//FC651	Send/Receive Schnittstelle
// ***************************************************************************
FUNCTION "FC_SR_QK" : VOID

TITLE =Send/Receive Empfang

AUTHOR: 	SIEMENS
FAMILY: 	SISTARS7
VERSION: 	4.02

//KNOW_HOW_PROTECT

// Datum	 Name			Aktion
// ---------------------------------------------------------------------------
// 19.05.99  Mahler		Neu



//Eingabeparameter
VAR_INPUT
	iFKT			: INT;		//Aufrufmodus
END_VAR

//Ausgabeparameter
//VAR_OUTPUT
//END_VAR


//Temporäre/Lokale Variable
VAR_TEMP

	anyQUEL	: ANY; 	         //Offset=0, Zeiger muss an erster Stelle stehen
	anyZIEL	: ANY;		   //Offset=10,
	uVerb		:"XC_INIT_SR_UDT";   //Offset=20


	iID		: INT;
	wLADDR	: WORD;

	boNDR		: BOOL;
	boDONE	: BOOL;
	boERROR	: BOOL;
	wSTATUS	: WORD;
	iLEN		: INT;

	iret		: INT;

 	iLoop	      : INT;
      iAct		: INT;

	dwPTR1      : DWORD;
	dwPTR2	: DWORD;
      dwOff		: DWORD;

	boSend	: BOOL;

	byPCU		: BYTE;
	bySavVB	: BYTE;

	bosec		: BOOL;
	bomin		: BOOL;
	iTSoll	: INT;
	iTIst		: INT;

END_VAR

BEGIN

NETWORK
TITLE = Vorbesetzen der Zeiger
// ===========================================================================
//Pionter fuer den Empfangspuffer zusammenstellen
//Any-Pointer:
//Byte 0	: S7-Typ 		= 16=10H                 LB0,LB10
//Byte 1	: Datentyp		= 02=Byte			 LB1,LB11
//Byte 2/3	: Wiederholungsfaktor				 LW2,LW12
//Byte 4/5	: DB-Nummer						 LW4,LW14
//Byte 6-9	: Bereichszeiger					 LD6,LD16

	L 16;		//S7-Typ
	T LB 0;
	T LB 10;
	L 2;		//Datentyp=Byte
	T LB1;
	T LB11;

	L "SYS".u.byAS;
      T  #byPCU;
	L "XC_VERB_SR".bPCU;		//Pruefen ob PCU-NR im Bereich 1 .. 16 veraendert
	==I;
      spb end1;
	l #byPCU;
	l 16;
	>I;
	spb end1;
	l #byPCU;
	T "XC_VERB_SR".bPCU;
      S "XC_VERB_SR".boINIT;
end1: nop 0;
NETWORK
TITLE =INIT	- Verbindungsblock vorbesetzen
// ===========================================================================
      l iFKT;
      l 1;
      <>I;
	spb end2;
	un "XC_VERB_SR".boINIT;
      SPB end2;
      R "XC_VERB_SR".boINIT;

//PCU-Nummer je nach eigener Nummer eintragen
      L  "XC_VERB_SR".iOffset;
      L 1;
      +I;
      sld 3;
      t #dwPtr1;						//Zeiger auf DBB fuer PCU z.B. 201 Aktiv
      L  "XC_VERB_SR".iOffset;
      L 7;
      +I;
      sld 3;
      t #dwPtr2;						//Zeiger auf DBB fuer PCU z.B. 207 Normal
      L  "XC_VERB_SR".iLen;
      sld 3;
	t #dwOff;

	AUF "XC_VERB_SR";

      L  #byPCU;			//Sprungleiste
      spl ende;
      spa Lo20;
      spa AS01;
      spa AS02;
      spa AS03;
      spa AS04;
      spa AS05;
      spa AS06;
      spa AS07;
      spa AS08;
      spa AS09;
      spa AS10;
      spa AS11;
      spa AS12;
      spa AS13;
      spa AS14;
      spa AS15;
      spa AS16;
ende:	spa Lo20;

AS01:	L 2; 							//Verbindung 1 PCU-NR eintragen
    	T  DBB[#dwPTR1];
	T  DBB[#dwPTR2];
      L  #dwOff;
      L  #dwPTR1;
      +D;
      T  #dwPTR1;
      L  #dwOff;
      L  #dwPTR2;
      +D;
      T  #dwPTR2;

	L 3; 							//Verbindung 2 PCU-NR eintragen
    	T  DBB[#dwPTR1];
	T  DBB[#dwPTR2];
      L  #dwOff;
      L  #dwPTR1;
      +D;
      T  #dwPTR1;
      L  #dwOff;
      L  #dwPTR2;
      +D;
      T  #dwPTR2;

	L 4; 							//Verbindung 3 PCU-NR eintragen
    	T  DBB[#dwPTR1];
	T  DBB[#dwPTR2];
      L  #dwOff;
      L  #dwPTR1;
      +D;
      T  #dwPTR1;
      L  #dwOff;
      L  #dwPTR2;
      +D;
      T  #dwPTR2;

	L 5; 							//Verbindung 4 PCU-NR eintragen
    	T  DBB[#dwPTR1];
	T  DBB[#dwPTR2];
      L  #dwOff;
      L  #dwPTR1;
      +D;
      T  #dwPTR1;
      L  #dwOff;
      L  #dwPTR2;
      +D;
      T  #dwPTR2;

	L 6; 							//Verbindung 5 PCU-NR eintragen
    	T  DBB[#dwPTR1];
	T  DBB[#dwPTR2];
      L  #dwOff;
      L  #dwPTR1;
      +D;
      T  #dwPTR1;
      L  #dwOff;
      L  #dwPTR2;
      +D;
      T  #dwPTR2;


	L 7; 							//Verbindung 6 PCU-NR eintragen
    	T  DBB[#dwPTR1];
	T  DBB[#dwPTR2];
      L  #dwOff;
      L  #dwPTR1;
      +D;
      T  #dwPTR1;
      L  #dwOff;
      L  #dwPTR2;
      +D;
      T  #dwPTR2;

	L 8; 							//Verbindung 7 PCU-NR eintragen
    	T  DBB[#dwPTR1];
	T  DBB[#dwPTR2];
      L  #dwOff;
      L  #dwPTR1;
      +D;
      T  #dwPTR1;
      L  #dwOff;
      L  #dwPTR2;
      +D;
      T  #dwPTR2;

	L 9; 							//Verbindung 8  PCU-NR eintragen
    	T  DBB[#dwPTR1];
	T  DBB[#dwPTR2];
      L  #dwOff;
      L  #dwPTR1;
      +D;
      T  #dwPTR1;
      L  #dwOff;
      L  #dwPTR2;
      +D;
      T  #dwPTR2;

	L 10; 						//Verbindung 9 PCU-NR eintragen
    	T  DBB[#dwPTR1];
	T  DBB[#dwPTR2];
      L  #dwOff;
      L  #dwPTR1;
      +D;
      T  #dwPTR1;
      L  #dwOff;
      L  #dwPTR2;
      +D;
      T  #dwPTR2;

	L 11; 						//Verbindung 10 PCU-NR eintragen
    	T  DBB[#dwPTR1];
	T  DBB[#dwPTR2];
      L  #dwOff;
      L  #dwPTR1;
      +D;
      T  #dwPTR1;
      L  #dwOff;
      L  #dwPTR2;
      +D;
      T  #dwPTR2;

	L 12; 						//Verbindung 11 PCU-NR eintragen
    	T  DBB[#dwPTR1];
	T  DBB[#dwPTR2];
      L  #dwOff;
      L  #dwPTR1;
      +D;
      T  #dwPTR1;
      L  #dwOff;
      L  #dwPTR2;
      +D;
      T  #dwPTR2;

	L 13; 						//Verbindung 12 PCU-NR eintragen
    	T  DBB[#dwPTR1];
	T  DBB[#dwPTR2];
      L  #dwOff;
      L  #dwPTR1;
      +D;
      T  #dwPTR1;
      L  #dwOff;
      L  #dwPTR2;
      +D;
      T  #dwPTR2;

	L 14; 						//Verbindung 13 PCU-NR eintragen
    	T  DBB[#dwPTR1];
	T  DBB[#dwPTR2];
      L  #dwOff;
      L  #dwPTR1;
      +D;
      T  #dwPTR1;
      L  #dwOff;
      L  #dwPTR2;
      +D;
      T  #dwPTR2;

	L 15; 						//Verbindung 14 PCU-NR eintragen
    	T  DBB[#dwPTR1];
	T  DBB[#dwPTR2];
      L  #dwOff;
      L  #dwPTR1;
      +D;
      T  #dwPTR1;
      L  #dwOff;
      L  #dwPTR2;
      +D;
      T  #dwPTR2;

	L 16; 						//Verbindung 15 PCU-NR eintragen
    	T  DBB[#dwPTR1];
	T  DBB[#dwPTR2];
      L  #dwOff;
      L  #dwPTR1;
      +D;
      T  #dwPTR1;
      L  #dwOff;
      L  #dwPTR2;
      +D;
      T  #dwPTR2;
	spa Lo20;

AS02:	L 1; 							//Verbindung 1 PCU-NR eintragen
    	T  DBB[#dwPTR1];
	T  DBB[#dwPTR2];
      L  #dwOff;
      L  #dwPTR1;
      +D;
      T  #dwPTR1;
      L  #dwOff;
      L  #dwPTR2;
      +D;
      T  #dwPTR2;

	L 16; 							//Verbindung 2 PCU-NR eintragen
    	T  DBB[#dwPTR1];
	T  DBB[#dwPTR2];
      L  #dwOff;
      L  #dwPTR1;
      +D;
      T  #dwPTR1;
      L  #dwOff;
      L  #dwPTR2;
      +D;
      T  #dwPTR2;

	L 3; 							//Verbindung 3 PCU-NR eintragen
    	T  DBB[#dwPTR1];
	T  DBB[#dwPTR2];
      L  #dwOff;
      L  #dwPTR1;
      +D;
      T  #dwPTR1;
      L  #dwOff;
      L  #dwPTR2;
      +D;
      T  #dwPTR2;

	L 4; 							//Verbindung 4 PCU-NR eintragen
    	T  DBB[#dwPTR1];
	T  DBB[#dwPTR2];
      L  #dwOff;
      L  #dwPTR1;
      +D;
      T  #dwPTR1;
      L  #dwOff;
      L  #dwPTR2;
      +D;
      T  #dwPTR2;

	L 5; 							//Verbindung 5 PCU-NR eintragen
    	T  DBB[#dwPTR1];
	T  DBB[#dwPTR2];
      L  #dwOff;
      L  #dwPTR1;
      +D;
      T  #dwPTR1;
      L  #dwOff;
      L  #dwPTR2;
      +D;
      T  #dwPTR2;


	L 6; 							//Verbindung 6 PCU-NR eintragen
    	T  DBB[#dwPTR1];
	T  DBB[#dwPTR2];
      L  #dwOff;
      L  #dwPTR1;
      +D;
      T  #dwPTR1;
      L  #dwOff;
      L  #dwPTR2;
      +D;
      T  #dwPTR2;

	L 7; 							//Verbindung 7 PCU-NR eintragen
    	T  DBB[#dwPTR1];
	T  DBB[#dwPTR2];
      L  #dwOff;
      L  #dwPTR1;
      +D;
      T  #dwPTR1;
      L  #dwOff;
      L  #dwPTR2;
      +D;
      T  #dwPTR2;

	L 8; 							//Verbindung 8  PCU-NR eintragen
    	T  DBB[#dwPTR1];
	T  DBB[#dwPTR2];
      L  #dwOff;
      L  #dwPTR1;
      +D;
      T  #dwPTR1;
      L  #dwOff;
      L  #dwPTR2;
      +D;
      T  #dwPTR2;

	L 9; 						//Verbindung 9 PCU-NR eintragen
    	T  DBB[#dwPTR1];
	T  DBB[#dwPTR2];
      L  #dwOff;
      L  #dwPTR1;
      +D;
      T  #dwPTR1;
      L  #dwOff;
      L  #dwPTR2;
      +D;
      T  #dwPTR2;

	L 10; 						//Verbindung 10 PCU-NR eintragen
    	T  DBB[#dwPTR1];
	T  DBB[#dwPTR2];
      L  #dwOff;
      L  #dwPTR1;
      +D;
      T  #dwPTR1;
      L  #dwOff;
      L  #dwPTR2;
      +D;
      T  #dwPTR2;

	L 11; 						//Verbindung 11 PCU-NR eintragen
    	T  DBB[#dwPTR1];
	T  DBB[#dwPTR2];
      L  #dwOff;
      L  #dwPTR1;
      +D;
      T  #dwPTR1;
      L  #dwOff;
      L  #dwPTR2;
      +D;
      T  #dwPTR2;

	L 12; 						//Verbindung 12 PCU-NR eintragen
    	T  DBB[#dwPTR1];
	T  DBB[#dwPTR2];
      L  #dwOff;
      L  #dwPTR1;
      +D;
      T  #dwPTR1;
      L  #dwOff;
      L  #dwPTR2;
      +D;
      T  #dwPTR2;

	L 13; 						//Verbindung 13 PCU-NR eintragen
    	T  DBB[#dwPTR1];
	T  DBB[#dwPTR2];
      L  #dwOff;
      L  #dwPTR1;
      +D;
      T  #dwPTR1;
      L  #dwOff;
      L  #dwPTR2;
      +D;
      T  #dwPTR2;

	L 14; 						//Verbindung 14 PCU-NR eintragen
    	T  DBB[#dwPTR1];
	T  DBB[#dwPTR2];
      L  #dwOff;
      L  #dwPTR1;
      +D;
      T  #dwPTR1;
      L  #dwOff;
      L  #dwPTR2;
      +D;
      T  #dwPTR2;

	L 15; 						//Verbindung 15 PCU-NR eintragen
    	T  DBB[#dwPTR1];
	T  DBB[#dwPTR2];
      L  #dwOff;
      L  #dwPTR1;
      +D;
      T  #dwPTR1;
      L  #dwOff;
      L  #dwPTR2;
      +D;
      T  #dwPTR2;
	spa Lo20;

AS03:	L 15; 							//Verbindung 1 PCU-NR eintragen
    	T  DBB[#dwPTR1];
	T  DBB[#dwPTR2];
      L  #dwOff;
      L  #dwPTR1;
      +D;
      T  #dwPTR1;
      L  #dwOff;
      L  #dwPTR2;
      +D;
      T  #dwPTR2;

	L 1; 							//Verbindung 2 PCU-NR eintragen
    	T  DBB[#dwPTR1];
	T  DBB[#dwPTR2];
      L  #dwOff;
      L  #dwPTR1;
      +D;
      T  #dwPTR1;
      L  #dwOff;
      L  #dwPTR2;
      +D;
      T  #dwPTR2;

	L 2; 							//Verbindung 3 PCU-NR eintragen
    	T  DBB[#dwPTR1];
	T  DBB[#dwPTR2];
      L  #dwOff;
      L  #dwPTR1;
      +D;
      T  #dwPTR1;
      L  #dwOff;
      L  #dwPTR2;
      +D;
      T  #dwPTR2;

	L 16; 							//Verbindung 4 PCU-NR eintragen
    	T  DBB[#dwPTR1];
	T  DBB[#dwPTR2];
      L  #dwOff;
      L  #dwPTR1;
      +D;
      T  #dwPTR1;
      L  #dwOff;
      L  #dwPTR2;
      +D;
      T  #dwPTR2;

	L 4; 							//Verbindung 5 PCU-NR eintragen
    	T  DBB[#dwPTR1];
	T  DBB[#dwPTR2];
      L  #dwOff;
      L  #dwPTR1;
      +D;
      T  #dwPTR1;
      L  #dwOff;
      L  #dwPTR2;
      +D;
      T  #dwPTR2;


	L 5; 							//Verbindung 6 PCU-NR eintragen
    	T  DBB[#dwPTR1];
	T  DBB[#dwPTR2];
      L  #dwOff;
      L  #dwPTR1;
      +D;
      T  #dwPTR1;
      L  #dwOff;
      L  #dwPTR2;
      +D;
      T  #dwPTR2;

	L 6; 							//Verbindung 7 PCU-NR eintragen
    	T  DBB[#dwPTR1];
	T  DBB[#dwPTR2];
      L  #dwOff;
      L  #dwPTR1;
      +D;
      T  #dwPTR1;
      L  #dwOff;
      L  #dwPTR2;
      +D;
      T  #dwPTR2;

	L 7; 							//Verbindung 8  PCU-NR eintragen
    	T  DBB[#dwPTR1];
	T  DBB[#dwPTR2];
      L  #dwOff;
      L  #dwPTR1;
      +D;
      T  #dwPTR1;
      L  #dwOff;
      L  #dwPTR2;
      +D;
      T  #dwPTR2;

	L 8; 						//Verbindung 9 PCU-NR eintragen
    	T  DBB[#dwPTR1];
	T  DBB[#dwPTR2];
      L  #dwOff;
      L  #dwPTR1;
      +D;
      T  #dwPTR1;
      L  #dwOff;
      L  #dwPTR2;
      +D;
      T  #dwPTR2;

	L 9; 						//Verbindung 10 PCU-NR eintragen
    	T  DBB[#dwPTR1];
	T  DBB[#dwPTR2];
      L  #dwOff;
      L  #dwPTR1;
      +D;
      T  #dwPTR1;
      L  #dwOff;
      L  #dwPTR2;
      +D;
      T  #dwPTR2;

	L 10; 						//Verbindung 11 PCU-NR eintragen
    	T  DBB[#dwPTR1];
	T  DBB[#dwPTR2];
      L  #dwOff;
      L  #dwPTR1;
      +D;
      T  #dwPTR1;
      L  #dwOff;
      L  #dwPTR2;
      +D;
      T  #dwPTR2;

	L 11; 						//Verbindung 12 PCU-NR eintragen
    	T  DBB[#dwPTR1];
	T  DBB[#dwPTR2];
      L  #dwOff;
      L  #dwPTR1;
      +D;
      T  #dwPTR1;
      L  #dwOff;
      L  #dwPTR2;
      +D;
      T  #dwPTR2;

	L 12; 						//Verbindung 13 PCU-NR eintragen
    	T  DBB[#dwPTR1];
	T  DBB[#dwPTR2];
      L  #dwOff;
      L  #dwPTR1;
      +D;
      T  #dwPTR1;
      L  #dwOff;
      L  #dwPTR2;
      +D;
      T  #dwPTR2;

	L 13; 						//Verbindung 14 PCU-NR eintragen
    	T  DBB[#dwPTR1];
	T  DBB[#dwPTR2];
      L  #dwOff;
      L  #dwPTR1;
      +D;
      T  #dwPTR1;
      L  #dwOff;
      L  #dwPTR2;
      +D;
      T  #dwPTR2;

	L 14; 						//Verbindung 15 PCU-NR eintragen
    	T  DBB[#dwPTR1];
	T  DBB[#dwPTR2];
      L  #dwOff;
      L  #dwPTR1;
      +D;
      T  #dwPTR1;
      L  #dwOff;
      L  #dwPTR2;
      +D;
      T  #dwPTR2;
	spa Lo20;

AS04:	L 14; 							//Verbindung 1 PCU-NR eintragen
    	T  DBB[#dwPTR1];
	T  DBB[#dwPTR2];
      L  #dwOff;
      L  #dwPTR1;
      +D;
      T  #dwPTR1;
      L  #dwOff;
      L  #dwPTR2;
      +D;
      T  #dwPTR2;

	L 15; 							//Verbindung 2 PCU-NR eintragen
    	T  DBB[#dwPTR1];
	T  DBB[#dwPTR2];
      L  #dwOff;
      L  #dwPTR1;
      +D;
      T  #dwPTR1;
      L  #dwOff;
      L  #dwPTR2;
      +D;
      T  #dwPTR2;

	L 1; 							//Verbindung 3 PCU-NR eintragen
    	T  DBB[#dwPTR1];
	T  DBB[#dwPTR2];
      L  #dwOff;
      L  #dwPTR1;
      +D;
      T  #dwPTR1;
      L  #dwOff;
      L  #dwPTR2;
      +D;
      T  #dwPTR2;

	L 2; 							//Verbindung 4 PCU-NR eintragen
    	T  DBB[#dwPTR1];
	T  DBB[#dwPTR2];
      L  #dwOff;
      L  #dwPTR1;
      +D;
      T  #dwPTR1;
      L  #dwOff;
      L  #dwPTR2;
      +D;
      T  #dwPTR2;

	L 3; 							//Verbindung 5 PCU-NR eintragen
    	T  DBB[#dwPTR1];
	T  DBB[#dwPTR2];
      L  #dwOff;
      L  #dwPTR1;
      +D;
      T  #dwPTR1;
      L  #dwOff;
      L  #dwPTR2;
      +D;
      T  #dwPTR2;


	L 16; 							//Verbindung 6 PCU-NR eintragen
    	T  DBB[#dwPTR1];
	T  DBB[#dwPTR2];
      L  #dwOff;
      L  #dwPTR1;
      +D;
      T  #dwPTR1;
      L  #dwOff;
      L  #dwPTR2;
      +D;
      T  #dwPTR2;

	L 5; 							//Verbindung 7 PCU-NR eintragen
    	T  DBB[#dwPTR1];
	T  DBB[#dwPTR2];
      L  #dwOff;
      L  #dwPTR1;
      +D;
      T  #dwPTR1;
      L  #dwOff;
      L  #dwPTR2;
      +D;
      T  #dwPTR2;

	L 6; 							//Verbindung 8  PCU-NR eintragen
    	T  DBB[#dwPTR1];
	T  DBB[#dwPTR2];
      L  #dwOff;
      L  #dwPTR1;
      +D;
      T  #dwPTR1;
      L  #dwOff;
      L  #dwPTR2;
      +D;
      T  #dwPTR2;

	L 7; 						//Verbindung 9 PCU-NR eintragen
    	T  DBB[#dwPTR1];
	T  DBB[#dwPTR2];
      L  #dwOff;
      L  #dwPTR1;
      +D;
      T  #dwPTR1;
      L  #dwOff;
      L  #dwPTR2;
      +D;
      T  #dwPTR2;

	L 8; 						//Verbindung 10 PCU-NR eintragen
    	T  DBB[#dwPTR1];
	T  DBB[#dwPTR2];
      L  #dwOff;
      L  #dwPTR1;
      +D;
      T  #dwPTR1;
      L  #dwOff;
      L  #dwPTR2;
      +D;
      T  #dwPTR2;

	L 9; 						//Verbindung 11 PCU-NR eintragen
    	T  DBB[#dwPTR1];
	T  DBB[#dwPTR2];
      L  #dwOff;
      L  #dwPTR1;
      +D;
      T  #dwPTR1;
      L  #dwOff;
      L  #dwPTR2;
      +D;
      T  #dwPTR2;

	L 10; 						//Verbindung 12 PCU-NR eintragen
    	T  DBB[#dwPTR1];
	T  DBB[#dwPTR2];
      L  #dwOff;
      L  #dwPTR1;
      +D;
      T  #dwPTR1;
      L  #dwOff;
      L  #dwPTR2;
      +D;
      T  #dwPTR2;

	L 11; 						//Verbindung 13 PCU-NR eintragen
    	T  DBB[#dwPTR1];
	T  DBB[#dwPTR2];
      L  #dwOff;
      L  #dwPTR1;
      +D;
      T  #dwPTR1;
      L  #dwOff;
      L  #dwPTR2;
      +D;
      T  #dwPTR2;

	L 12; 						//Verbindung 14 PCU-NR eintragen
    	T  DBB[#dwPTR1];
	T  DBB[#dwPTR2];
      L  #dwOff;
      L  #dwPTR1;
      +D;
      T  #dwPTR1;
      L  #dwOff;
      L  #dwPTR2;
      +D;
      T  #dwPTR2;

	L 13; 						//Verbindung 15 PCU-NR eintragen
    	T  DBB[#dwPTR1];
	T  DBB[#dwPTR2];
      L  #dwOff;
      L  #dwPTR1;
      +D;
      T  #dwPTR1;
      L  #dwOff;
      L  #dwPTR2;
      +D;
      T  #dwPTR2;
	spa Lo20;

AS05:	L 13; 							//Verbindung 1 PCU-NR eintragen
    	T  DBB[#dwPTR1];
	T  DBB[#dwPTR2];
      L  #dwOff;
      L  #dwPTR1;
      +D;
      T  #dwPTR1;
      L  #dwOff;
      L  #dwPTR2;
      +D;
      T  #dwPTR2;

	L 14; 							//Verbindung 2 PCU-NR eintragen
    	T  DBB[#dwPTR1];
	T  DBB[#dwPTR2];
      L  #dwOff;
      L  #dwPTR1;
      +D;
      T  #dwPTR1;
      L  #dwOff;
      L  #dwPTR2;
      +D;
      T  #dwPTR2;

	L 15; 							//Verbindung 3 PCU-NR eintragen
    	T  DBB[#dwPTR1];
	T  DBB[#dwPTR2];
      L  #dwOff;
      L  #dwPTR1;
      +D;
      T  #dwPTR1;
      L  #dwOff;
      L  #dwPTR2;
      +D;
      T  #dwPTR2;

	L 1; 							//Verbindung 4 PCU-NR eintragen
    	T  DBB[#dwPTR1];
	T  DBB[#dwPTR2];
      L  #dwOff;
      L  #dwPTR1;
      +D;
      T  #dwPTR1;
      L  #dwOff;
      L  #dwPTR2;
      +D;
      T  #dwPTR2;

	L 2; 							//Verbindung 5 PCU-NR eintragen
    	T  DBB[#dwPTR1];
	T  DBB[#dwPTR2];
      L  #dwOff;
      L  #dwPTR1;
      +D;
      T  #dwPTR1;
      L  #dwOff;
      L  #dwPTR2;
      +D;
      T  #dwPTR2;


	L 3; 							//Verbindung 6 PCU-NR eintragen
    	T  DBB[#dwPTR1];
	T  DBB[#dwPTR2];
      L  #dwOff;
      L  #dwPTR1;
      +D;
      T  #dwPTR1;
      L  #dwOff;
      L  #dwPTR2;
      +D;
      T  #dwPTR2;

	L 4; 							//Verbindung 7 PCU-NR eintragen
    	T  DBB[#dwPTR1];
	T  DBB[#dwPTR2];
      L  #dwOff;
      L  #dwPTR1;
      +D;
      T  #dwPTR1;
      L  #dwOff;
      L  #dwPTR2;
      +D;
      T  #dwPTR2;

	L 16; 							//Verbindung 8  PCU-NR eintragen
    	T  DBB[#dwPTR1];
	T  DBB[#dwPTR2];
      L  #dwOff;
      L  #dwPTR1;
      +D;
      T  #dwPTR1;
      L  #dwOff;
      L  #dwPTR2;
      +D;
      T  #dwPTR2;

	L 6; 						//Verbindung 9 PCU-NR eintragen
    	T  DBB[#dwPTR1];
	T  DBB[#dwPTR2];
      L  #dwOff;
      L  #dwPTR1;
      +D;
      T  #dwPTR1;
      L  #dwOff;
      L  #dwPTR2;
      +D;
      T  #dwPTR2;

	L 7; 						//Verbindung 10 PCU-NR eintragen
    	T  DBB[#dwPTR1];
	T  DBB[#dwPTR2];
      L  #dwOff;
      L  #dwPTR1;
      +D;
      T  #dwPTR1;
      L  #dwOff;
      L  #dwPTR2;
      +D;
      T  #dwPTR2;

	L 8; 						//Verbindung 11 PCU-NR eintragen
    	T  DBB[#dwPTR1];
	T  DBB[#dwPTR2];
      L  #dwOff;
      L  #dwPTR1;
      +D;
      T  #dwPTR1;
      L  #dwOff;
      L  #dwPTR2;
      +D;
      T  #dwPTR2;

	L 9; 						//Verbindung 12 PCU-NR eintragen
    	T  DBB[#dwPTR1];
	T  DBB[#dwPTR2];
      L  #dwOff;
      L  #dwPTR1;
      +D;
      T  #dwPTR1;
      L  #dwOff;
      L  #dwPTR2;
      +D;
      T  #dwPTR2;

	L 10; 						//Verbindung 13 PCU-NR eintragen
    	T  DBB[#dwPTR1];
	T  DBB[#dwPTR2];
      L  #dwOff;
      L  #dwPTR1;
      +D;
      T  #dwPTR1;
      L  #dwOff;
      L  #dwPTR2;
      +D;
      T  #dwPTR2;

	L 11;						//Verbindung 14 PCU-NR eintragen
    	T  DBB[#dwPTR1];
	T  DBB[#dwPTR2];
      L  #dwOff;
      L  #dwPTR1;
      +D;
      T  #dwPTR1;
      L  #dwOff;
      L  #dwPTR2;
      +D;
      T  #dwPTR2;

	L 12;						//Verbindung 15 PCU-NR eintragen
    	T  DBB[#dwPTR1];
	T  DBB[#dwPTR2];
      L  #dwOff;
      L  #dwPTR1;
      +D;
      T  #dwPTR1;
      L  #dwOff;
      L  #dwPTR2;
      +D;
      T  #dwPTR2;
	spa Lo20;

AS06:	L 12; 							//Verbindung 1 PCU-NR eintragen
    	T  DBB[#dwPTR1];
	T  DBB[#dwPTR2];
      L  #dwOff;
      L  #dwPTR1;
      +D;
      T  #dwPTR1;
      L  #dwOff;
      L  #dwPTR2;
      +D;
      T  #dwPTR2;

	L 13; 							//Verbindung 2 PCU-NR eintragen
    	T  DBB[#dwPTR1];
	T  DBB[#dwPTR2];
      L  #dwOff;
      L  #dwPTR1;
      +D;
      T  #dwPTR1;
      L  #dwOff;
      L  #dwPTR2;
      +D;
      T  #dwPTR2;

	L 14; 							//Verbindung 3 PCU-NR eintragen
    	T  DBB[#dwPTR1];
	T  DBB[#dwPTR2];
      L  #dwOff;
      L  #dwPTR1;
      +D;
      T  #dwPTR1;
      L  #dwOff;
      L  #dwPTR2;
      +D;
      T  #dwPTR2;

	L 15; 							//Verbindung 4 PCU-NR eintragen
    	T  DBB[#dwPTR1];
	T  DBB[#dwPTR2];
      L  #dwOff;
      L  #dwPTR1;
      +D;
      T  #dwPTR1;
      L  #dwOff;
      L  #dwPTR2;
      +D;
      T  #dwPTR2;

	L 1; 							//Verbindung 5 PCU-NR eintragen
    	T  DBB[#dwPTR1];
	T  DBB[#dwPTR2];
      L  #dwOff;
      L  #dwPTR1;
      +D;
      T  #dwPTR1;
      L  #dwOff;
      L  #dwPTR2;
      +D;
      T  #dwPTR2;


	L 2; 							//Verbindung 6 PCU-NR eintragen
    	T  DBB[#dwPTR1];
	T  DBB[#dwPTR2];
      L  #dwOff;
      L  #dwPTR1;
      +D;
      T  #dwPTR1;
      L  #dwOff;
      L  #dwPTR2;
      +D;
      T  #dwPTR2;

	L 3; 							//Verbindung 7 PCU-NR eintragen
    	T  DBB[#dwPTR1];
	T  DBB[#dwPTR2];
      L  #dwOff;
      L  #dwPTR1;
      +D;
      T  #dwPTR1;
      L  #dwOff;
      L  #dwPTR2;
      +D;
      T  #dwPTR2;

	L 4; 							//Verbindung 8  PCU-NR eintragen
    	T  DBB[#dwPTR1];
	T  DBB[#dwPTR2];
      L  #dwOff;
      L  #dwPTR1;
      +D;
      T  #dwPTR1;
      L  #dwOff;
      L  #dwPTR2;
      +D;
      T  #dwPTR2;

	L 5; 						//Verbindung 9 PCU-NR eintragen
    	T  DBB[#dwPTR1];
	T  DBB[#dwPTR2];
      L  #dwOff;
      L  #dwPTR1;
      +D;
      T  #dwPTR1;
      L  #dwOff;
      L  #dwPTR2;
      +D;
      T  #dwPTR2;

	L 16; 						//Verbindung 10 PCU-NR eintragen
    	T  DBB[#dwPTR1];
	T  DBB[#dwPTR2];
      L  #dwOff;
      L  #dwPTR1;
      +D;
      T  #dwPTR1;
      L  #dwOff;
      L  #dwPTR2;
      +D;
      T  #dwPTR2;

	L 7; 						//Verbindung 11 PCU-NR eintragen
    	T  DBB[#dwPTR1];
	T  DBB[#dwPTR2];
      L  #dwOff;
      L  #dwPTR1;
      +D;
      T  #dwPTR1;
      L  #dwOff;
      L  #dwPTR2;
      +D;
      T  #dwPTR2;

	L 8; 						//Verbindung 12 PCU-NR eintragen
    	T  DBB[#dwPTR1];
	T  DBB[#dwPTR2];
      L  #dwOff;
      L  #dwPTR1;
      +D;
      T  #dwPTR1;
      L  #dwOff;
      L  #dwPTR2;
      +D;
      T  #dwPTR2;

	L 9; 						//Verbindung 13 PCU-NR eintragen
    	T  DBB[#dwPTR1];
	T  DBB[#dwPTR2];
      L  #dwOff;
      L  #dwPTR1;
      +D;
      T  #dwPTR1;
      L  #dwOff;
      L  #dwPTR2;
      +D;
      T  #dwPTR2;

	L 10; 						//Verbindung 14 PCU-NR eintragen
    	T  DBB[#dwPTR1];
	T  DBB[#dwPTR2];
      L  #dwOff;
      L  #dwPTR1;
      +D;
      T  #dwPTR1;
      L  #dwOff;
      L  #dwPTR2;
      +D;
      T  #dwPTR2;

	L 11; 						//Verbindung 15 PCU-NR eintragen
    	T  DBB[#dwPTR1];
	T  DBB[#dwPTR2];
      L  #dwOff;
      L  #dwPTR1;
      +D;
      T  #dwPTR1;
      L  #dwOff;
      L  #dwPTR2;
      +D;
      T  #dwPTR2;
	spa Lo20;

AS07:	L 11; 							//Verbindung 1 PCU-NR eintragen
    	T  DBB[#dwPTR1];
	T  DBB[#dwPTR2];
      L  #dwOff;
      L  #dwPTR1;
      +D;
      T  #dwPTR1;
      L  #dwOff;
      L  #dwPTR2;
      +D;
      T  #dwPTR2;

	L 12; 							//Verbindung 2 PCU-NR eintragen
    	T  DBB[#dwPTR1];
	T  DBB[#dwPTR2];
      L  #dwOff;
      L  #dwPTR1;
      +D;
      T  #dwPTR1;
      L  #dwOff;
      L  #dwPTR2;
      +D;
      T  #dwPTR2;

	L 13; 							//Verbindung 3 PCU-NR eintragen
    	T  DBB[#dwPTR1];
	T  DBB[#dwPTR2];
      L  #dwOff;
      L  #dwPTR1;
      +D;
      T  #dwPTR1;
      L  #dwOff;
      L  #dwPTR2;
      +D;
      T  #dwPTR2;

	L 14; 							//Verbindung 4 PCU-NR eintragen
    	T  DBB[#dwPTR1];
	T  DBB[#dwPTR2];
      L  #dwOff;
      L  #dwPTR1;
      +D;
      T  #dwPTR1;
      L  #dwOff;
      L  #dwPTR2;
      +D;
      T  #dwPTR2;

	L 15; 							//Verbindung 5 PCU-NR eintragen
    	T  DBB[#dwPTR1];
	T  DBB[#dwPTR2];
      L  #dwOff;
      L  #dwPTR1;
      +D;
      T  #dwPTR1;
      L  #dwOff;
      L  #dwPTR2;
      +D;
      T  #dwPTR2;


	L 1; 							//Verbindung 6 PCU-NR eintragen
    	T  DBB[#dwPTR1];
	T  DBB[#dwPTR2];
      L  #dwOff;
      L  #dwPTR1;
      +D;
      T  #dwPTR1;
      L  #dwOff;
      L  #dwPTR2;
      +D;
      T  #dwPTR2;

	L 2; 							//Verbindung 7 PCU-NR eintragen
    	T  DBB[#dwPTR1];
	T  DBB[#dwPTR2];
      L  #dwOff;
      L  #dwPTR1;
      +D;
      T  #dwPTR1;
      L  #dwOff;
      L  #dwPTR2;
      +D;
      T  #dwPTR2;

	L 3; 							//Verbindung 8  PCU-NR eintragen
    	T  DBB[#dwPTR1];
	T  DBB[#dwPTR2];
      L  #dwOff;
      L  #dwPTR1;
      +D;
      T  #dwPTR1;
      L  #dwOff;
      L  #dwPTR2;
      +D;
      T  #dwPTR2;

	L 4; 						//Verbindung 9 PCU-NR eintragen
    	T  DBB[#dwPTR1];
	T  DBB[#dwPTR2];
      L  #dwOff;
      L  #dwPTR1;
      +D;
      T  #dwPTR1;
      L  #dwOff;
      L  #dwPTR2;
      +D;
      T  #dwPTR2;

	L 5; 						//Verbindung 10 PCU-NR eintragen
    	T  DBB[#dwPTR1];
	T  DBB[#dwPTR2];
      L  #dwOff;
      L  #dwPTR1;
      +D;
      T  #dwPTR1;
      L  #dwOff;
      L  #dwPTR2;
      +D;
      T  #dwPTR2;

	L 6; 						//Verbindung 11 PCU-NR eintragen
    	T  DBB[#dwPTR1];
	T  DBB[#dwPTR2];
      L  #dwOff;
      L  #dwPTR1;
      +D;
      T  #dwPTR1;
      L  #dwOff;
      L  #dwPTR2;
      +D;
      T  #dwPTR2;

	L 16; 						//Verbindung 12 PCU-NR eintragen
    	T  DBB[#dwPTR1];
	T  DBB[#dwPTR2];
      L  #dwOff;
      L  #dwPTR1;
      +D;
      T  #dwPTR1;
      L  #dwOff;
      L  #dwPTR2;
      +D;
      T  #dwPTR2;

	L 8; 						//Verbindung 13 PCU-NR eintragen
    	T  DBB[#dwPTR1];
	T  DBB[#dwPTR2];
      L  #dwOff;
      L  #dwPTR1;
      +D;
      T  #dwPTR1;
      L  #dwOff;
      L  #dwPTR2;
      +D;
      T  #dwPTR2;

	L 9; 						//Verbindung 14 PCU-NR eintragen
    	T  DBB[#dwPTR1];
	T  DBB[#dwPTR2];
      L  #dwOff;
      L  #dwPTR1;
      +D;
      T  #dwPTR1;
      L  #dwOff;
      L  #dwPTR2;
      +D;
      T  #dwPTR2;

	L 10; 						//Verbindung 15 PCU-NR eintragen
    	T  DBB[#dwPTR1];
	T  DBB[#dwPTR2];
      L  #dwOff;
      L  #dwPTR1;
      +D;
      T  #dwPTR1;
      L  #dwOff;
      L  #dwPTR2;
      +D;
      T  #dwPTR2;
	spa Lo20;

AS08:	L 10; 							//Verbindung 1 PCU-NR eintragen
    	T  DBB[#dwPTR1];
	T  DBB[#dwPTR2];
      L  #dwOff;
      L  #dwPTR1;
      +D;
      T  #dwPTR1;
      L  #dwOff;
      L  #dwPTR2;
      +D;
      T  #dwPTR2;

	L 11; 							//Verbindung 2 PCU-NR eintragen
    	T  DBB[#dwPTR1];
	T  DBB[#dwPTR2];
      L  #dwOff;
      L  #dwPTR1;
      +D;
      T  #dwPTR1;
      L  #dwOff;
      L  #dwPTR2;
      +D;
      T  #dwPTR2;

	L 12; 							//Verbindung 3 PCU-NR eintragen
    	T  DBB[#dwPTR1];
	T  DBB[#dwPTR2];
      L  #dwOff;
      L  #dwPTR1;
      +D;
      T  #dwPTR1;
      L  #dwOff;
      L  #dwPTR2;
      +D;
      T  #dwPTR2;

	L 13; 							//Verbindung 4 PCU-NR eintragen
    	T  DBB[#dwPTR1];
	T  DBB[#dwPTR2];
      L  #dwOff;
      L  #dwPTR1;
      +D;
      T  #dwPTR1;
      L  #dwOff;
      L  #dwPTR2;
      +D;
      T  #dwPTR2;

	L 14; 							//Verbindung 5 PCU-NR eintragen
    	T  DBB[#dwPTR1];
	T  DBB[#dwPTR2];
      L  #dwOff;
      L  #dwPTR1;
      +D;
      T  #dwPTR1;
      L  #dwOff;
      L  #dwPTR2;
      +D;
      T  #dwPTR2;


	L 15; 							//Verbindung 6 PCU-NR eintragen
    	T  DBB[#dwPTR1];
	T  DBB[#dwPTR2];
      L  #dwOff;
      L  #dwPTR1;
      +D;
      T  #dwPTR1;
      L  #dwOff;
      L  #dwPTR2;
      +D;
      T  #dwPTR2;

	L 1; 							//Verbindung 7 PCU-NR eintragen
    	T  DBB[#dwPTR1];
	T  DBB[#dwPTR2];
      L  #dwOff;
      L  #dwPTR1;
      +D;
      T  #dwPTR1;
      L  #dwOff;
      L  #dwPTR2;
      +D;
      T  #dwPTR2;

	L 2; 							//Verbindung 8  PCU-NR eintragen
    	T  DBB[#dwPTR1];
	T  DBB[#dwPTR2];
      L  #dwOff;
      L  #dwPTR1;
      +D;
      T  #dwPTR1;
      L  #dwOff;
      L  #dwPTR2;
      +D;
      T  #dwPTR2;

	L 3; 						//Verbindung 9 PCU-NR eintragen
    	T  DBB[#dwPTR1];
	T  DBB[#dwPTR2];
      L  #dwOff;
      L  #dwPTR1;
      +D;
      T  #dwPTR1;
      L  #dwOff;
      L  #dwPTR2;
      +D;
      T  #dwPTR2;

	L 4; 						//Verbindung 10 PCU-NR eintragen
    	T  DBB[#dwPTR1];
	T  DBB[#dwPTR2];
      L  #dwOff;
      L  #dwPTR1;
      +D;
      T  #dwPTR1;
      L  #dwOff;
      L  #dwPTR2;
      +D;
      T  #dwPTR2;

	L 5; 						//Verbindung 11 PCU-NR eintragen
    	T  DBB[#dwPTR1];
	T  DBB[#dwPTR2];
      L  #dwOff;
      L  #dwPTR1;
      +D;
      T  #dwPTR1;
      L  #dwOff;
      L  #dwPTR2;
      +D;
      T  #dwPTR2;

	L 6; 						//Verbindung 12 PCU-NR eintragen
    	T  DBB[#dwPTR1];
	T  DBB[#dwPTR2];
      L  #dwOff;
      L  #dwPTR1;
      +D;
      T  #dwPTR1;
      L  #dwOff;
      L  #dwPTR2;
      +D;
      T  #dwPTR2;

	L 7; 						//Verbindung 13 PCU-NR eintragen
    	T  DBB[#dwPTR1];
	T  DBB[#dwPTR2];
      L  #dwOff;
      L  #dwPTR1;
      +D;
      T  #dwPTR1;
      L  #dwOff;
      L  #dwPTR2;
      +D;
      T  #dwPTR2;

	L 16; 						//Verbindung 14 PCU-NR eintragen
    	T  DBB[#dwPTR1];
	T  DBB[#dwPTR2];
      L  #dwOff;
      L  #dwPTR1;
      +D;
      T  #dwPTR1;
      L  #dwOff;
      L  #dwPTR2;
      +D;
      T  #dwPTR2;

	L 9; 						//Verbindung 15 PCU-NR eintragen
    	T  DBB[#dwPTR1];
	T  DBB[#dwPTR2];
      L  #dwOff;
      L  #dwPTR1;
      +D;
      T  #dwPTR1;
      L  #dwOff;
      L  #dwPTR2;
      +D;
      T  #dwPTR2;
	spa Lo20;

AS09:	L 16; 							//Verbindung 1 PCU-NR eintragen
    	T  DBB[#dwPTR1];
	T  DBB[#dwPTR2];
      L  #dwOff;
      L  #dwPTR1;
      +D;
      T  #dwPTR1;
      L  #dwOff;
      L  #dwPTR2;
      +D;
      T  #dwPTR2;

	L 10; 							//Verbindung 2 PCU-NR eintragen
    	T  DBB[#dwPTR1];
	T  DBB[#dwPTR2];
      L  #dwOff;
      L  #dwPTR1;
      +D;
      T  #dwPTR1;
      L  #dwOff;
      L  #dwPTR2;
      +D;
      T  #dwPTR2;

	L 11; 							//Verbindung 3 PCU-NR eintragen
    	T  DBB[#dwPTR1];
	T  DBB[#dwPTR2];
      L  #dwOff;
      L  #dwPTR1;
      +D;
      T  #dwPTR1;
      L  #dwOff;
      L  #dwPTR2;
      +D;
      T  #dwPTR2;

	L 12; 							//Verbindung 4 PCU-NR eintragen
    	T  DBB[#dwPTR1];
	T  DBB[#dwPTR2];
      L  #dwOff;
      L  #dwPTR1;
      +D;
      T  #dwPTR1;
      L  #dwOff;
      L  #dwPTR2;
      +D;
      T  #dwPTR2;

	L 13; 							//Verbindung 5 PCU-NR eintragen
    	T  DBB[#dwPTR1];
	T  DBB[#dwPTR2];
      L  #dwOff;
      L  #dwPTR1;
      +D;
      T  #dwPTR1;
      L  #dwOff;
      L  #dwPTR2;
      +D;
      T  #dwPTR2;


	L 14; 							//Verbindung 6 PCU-NR eintragen
    	T  DBB[#dwPTR1];
	T  DBB[#dwPTR2];
      L  #dwOff;
      L  #dwPTR1;
      +D;
      T  #dwPTR1;
      L  #dwOff;
      L  #dwPTR2;
      +D;
      T  #dwPTR2;

	L 15; 							//Verbindung 7 PCU-NR eintragen
    	T  DBB[#dwPTR1];
	T  DBB[#dwPTR2];
      L  #dwOff;
      L  #dwPTR1;
      +D;
      T  #dwPTR1;
      L  #dwOff;
      L  #dwPTR2;
      +D;
      T  #dwPTR2;

	L 1; 							//Verbindung 8  PCU-NR eintragen
    	T  DBB[#dwPTR1];
	T  DBB[#dwPTR2];
      L  #dwOff;
      L  #dwPTR1;
      +D;
      T  #dwPTR1;
      L  #dwOff;
      L  #dwPTR2;
      +D;
      T  #dwPTR2;

	L 2; 						//Verbindung 9 PCU-NR eintragen
    	T  DBB[#dwPTR1];
	T  DBB[#dwPTR2];
      L  #dwOff;
      L  #dwPTR1;
      +D;
      T  #dwPTR1;
      L  #dwOff;
      L  #dwPTR2;
      +D;
      T  #dwPTR2;

	L 3; 						//Verbindung 10 PCU-NR eintragen
    	T  DBB[#dwPTR1];
	T  DBB[#dwPTR2];
      L  #dwOff;
      L  #dwPTR1;
      +D;
      T  #dwPTR1;
      L  #dwOff;
      L  #dwPTR2;
      +D;
      T  #dwPTR2;

	L 4; 						//Verbindung 11 PCU-NR eintragen
    	T  DBB[#dwPTR1];
	T  DBB[#dwPTR2];
      L  #dwOff;
      L  #dwPTR1;
      +D;
      T  #dwPTR1;
      L  #dwOff;
      L  #dwPTR2;
      +D;
      T  #dwPTR2;

	L 5; 						//Verbindung 12 PCU-NR eintragen
    	T  DBB[#dwPTR1];
	T  DBB[#dwPTR2];
      L  #dwOff;
      L  #dwPTR1;
      +D;
      T  #dwPTR1;
      L  #dwOff;
      L  #dwPTR2;
      +D;
      T  #dwPTR2;

	L 6; 						//Verbindung 13 PCU-NR eintragen
    	T  DBB[#dwPTR1];
	T  DBB[#dwPTR2];
      L  #dwOff;
      L  #dwPTR1;
      +D;
      T  #dwPTR1;
      L  #dwOff;
      L  #dwPTR2;
      +D;
      T  #dwPTR2;

	L 7; 						//Verbindung 14 PCU-NR eintragen
    	T  DBB[#dwPTR1];
	T  DBB[#dwPTR2];
      L  #dwOff;
      L  #dwPTR1;
      +D;
      T  #dwPTR1;
      L  #dwOff;
      L  #dwPTR2;
      +D;
      T  #dwPTR2;

	L 8; 						//Verbindung 15 PCU-NR eintragen
    	T  DBB[#dwPTR1];
	T  DBB[#dwPTR2];
      L  #dwOff;
      L  #dwPTR1;
      +D;
      T  #dwPTR1;
      L  #dwOff;
      L  #dwPTR2;
      +D;
      T  #dwPTR2;
	spa Lo20;

AS10:	L 8; 							//Verbindung 1 PCU-NR eintragen
    	T  DBB[#dwPTR1];
	T  DBB[#dwPTR2];
      L  #dwOff;
      L  #dwPTR1;
      +D;
      T  #dwPTR1;
      L  #dwOff;
      L  #dwPTR2;
      +D;
      T  #dwPTR2;

	L 9; 							//Verbindung 2 PCU-NR eintragen
    	T  DBB[#dwPTR1];
	T  DBB[#dwPTR2];
      L  #dwOff;
      L  #dwPTR1;
      +D;
      T  #dwPTR1;
      L  #dwOff;
      L  #dwPTR2;
      +D;
      T  #dwPTR2;

	L 16; 							//Verbindung 3 PCU-NR eintragen
    	T  DBB[#dwPTR1];
	T  DBB[#dwPTR2];
      L  #dwOff;
      L  #dwPTR1;
      +D;
      T  #dwPTR1;
      L  #dwOff;
      L  #dwPTR2;
      +D;
      T  #dwPTR2;

	L 11; 							//Verbindung 4 PCU-NR eintragen
    	T  DBB[#dwPTR1];
	T  DBB[#dwPTR2];
      L  #dwOff;
      L  #dwPTR1;
      +D;
      T  #dwPTR1;
      L  #dwOff;
      L  #dwPTR2;
      +D;
      T  #dwPTR2;

	L 12; 							//Verbindung 5 PCU-NR eintragen
    	T  DBB[#dwPTR1];
	T  DBB[#dwPTR2];
      L  #dwOff;
      L  #dwPTR1;
      +D;
      T  #dwPTR1;
      L  #dwOff;
      L  #dwPTR2;
      +D;
      T  #dwPTR2;


	L 13; 							//Verbindung 6 PCU-NR eintragen
    	T  DBB[#dwPTR1];
	T  DBB[#dwPTR2];
      L  #dwOff;
      L  #dwPTR1;
      +D;
      T  #dwPTR1;
      L  #dwOff;
      L  #dwPTR2;
      +D;
      T  #dwPTR2;

	L 14; 							//Verbindung 7 PCU-NR eintragen
    	T  DBB[#dwPTR1];
	T  DBB[#dwPTR2];
      L  #dwOff;
      L  #dwPTR1;
      +D;
      T  #dwPTR1;
      L  #dwOff;
      L  #dwPTR2;
      +D;
      T  #dwPTR2;

	L 15; 							//Verbindung 8  PCU-NR eintragen
    	T  DBB[#dwPTR1];
	T  DBB[#dwPTR2];
      L  #dwOff;
      L  #dwPTR1;
      +D;
      T  #dwPTR1;
      L  #dwOff;
      L  #dwPTR2;
      +D;
      T  #dwPTR2;

	L 1; 						//Verbindung 9 PCU-NR eintragen
    	T  DBB[#dwPTR1];
	T  DBB[#dwPTR2];
      L  #dwOff;
      L  #dwPTR1;
      +D;
      T  #dwPTR1;
      L  #dwOff;
      L  #dwPTR2;
      +D;
      T  #dwPTR2;

	L 2; 						//Verbindung 10 PCU-NR eintragen
    	T  DBB[#dwPTR1];
	T  DBB[#dwPTR2];
      L  #dwOff;
      L  #dwPTR1;
      +D;
      T  #dwPTR1;
      L  #dwOff;
      L  #dwPTR2;
      +D;
      T  #dwPTR2;

	L 3; 						//Verbindung 11 PCU-NR eintragen
    	T  DBB[#dwPTR1];
	T  DBB[#dwPTR2];
      L  #dwOff;
      L  #dwPTR1;
      +D;
      T  #dwPTR1;
      L  #dwOff;
      L  #dwPTR2;
      +D;
      T  #dwPTR2;

	L 4; 						//Verbindung 12 PCU-NR eintragen
    	T  DBB[#dwPTR1];
	T  DBB[#dwPTR2];
      L  #dwOff;
      L  #dwPTR1;
      +D;
      T  #dwPTR1;
      L  #dwOff;
      L  #dwPTR2;
      +D;
      T  #dwPTR2;

	L 5; 						//Verbindung 13 PCU-NR eintragen
    	T  DBB[#dwPTR1];
	T  DBB[#dwPTR2];
      L  #dwOff;
      L  #dwPTR1;
      +D;
      T  #dwPTR1;
      L  #dwOff;
      L  #dwPTR2;
      +D;
      T  #dwPTR2;

	L 6; 						//Verbindung 14 PCU-NR eintragen
    	T  DBB[#dwPTR1];
	T  DBB[#dwPTR2];
      L  #dwOff;
      L  #dwPTR1;
      +D;
      T  #dwPTR1;
      L  #dwOff;
      L  #dwPTR2;
      +D;
      T  #dwPTR2;

	L 7; 						//Verbindung 15 PCU-NR eintragen
    	T  DBB[#dwPTR1];
	T  DBB[#dwPTR2];
      L  #dwOff;
      L  #dwPTR1;
      +D;
      T  #dwPTR1;
      L  #dwOff;
      L  #dwPTR2;
      +D;
      T  #dwPTR2;
	spa Lo20;

AS11:	L 7; 							//Verbindung 1 PCU-NR eintragen
    	T  DBB[#dwPTR1];
	T  DBB[#dwPTR2];
      L  #dwOff;
      L  #dwPTR1;
      +D;
      T  #dwPTR1;
      L  #dwOff;
      L  #dwPTR2;
      +D;
      T  #dwPTR2;

	L 8; 							//Verbindung 2 PCU-NR eintragen
    	T  DBB[#dwPTR1];
	T  DBB[#dwPTR2];
      L  #dwOff;
      L  #dwPTR1;
      +D;
      T  #dwPTR1;
      L  #dwOff;
      L  #dwPTR2;
      +D;
      T  #dwPTR2;

	L 9; 							//Verbindung 3 PCU-NR eintragen
    	T  DBB[#dwPTR1];
	T  DBB[#dwPTR2];
      L  #dwOff;
      L  #dwPTR1;
      +D;
      T  #dwPTR1;
      L  #dwOff;
      L  #dwPTR2;
      +D;
      T  #dwPTR2;

	L 10; 							//Verbindung 4 PCU-NR eintragen
    	T  DBB[#dwPTR1];
	T  DBB[#dwPTR2];
      L  #dwOff;
      L  #dwPTR1;
      +D;
      T  #dwPTR1;
      L  #dwOff;
      L  #dwPTR2;
      +D;
      T  #dwPTR2;

	L 16; 							//Verbindung 5 PCU-NR eintragen
    	T  DBB[#dwPTR1];
	T  DBB[#dwPTR2];
      L  #dwOff;
      L  #dwPTR1;
      +D;
      T  #dwPTR1;
      L  #dwOff;
      L  #dwPTR2;
      +D;
      T  #dwPTR2;


	L 12; 							//Verbindung 6 PCU-NR eintragen
    	T  DBB[#dwPTR1];
	T  DBB[#dwPTR2];
      L  #dwOff;
      L  #dwPTR1;
      +D;
      T  #dwPTR1;
      L  #dwOff;
      L  #dwPTR2;
      +D;
      T  #dwPTR2;

	L 13; 							//Verbindung 7 PCU-NR eintragen
    	T  DBB[#dwPTR1];
	T  DBB[#dwPTR2];
      L  #dwOff;
      L  #dwPTR1;
      +D;
      T  #dwPTR1;
      L  #dwOff;
      L  #dwPTR2;
      +D;
      T  #dwPTR2;

	L 14; 							//Verbindung 8  PCU-NR eintragen
    	T  DBB[#dwPTR1];
	T  DBB[#dwPTR2];
      L  #dwOff;
      L  #dwPTR1;
      +D;
      T  #dwPTR1;
      L  #dwOff;
      L  #dwPTR2;
      +D;
      T  #dwPTR2;

	L 15; 						//Verbindung 9 PCU-NR eintragen
    	T  DBB[#dwPTR1];
	T  DBB[#dwPTR2];
      L  #dwOff;
      L  #dwPTR1;
      +D;
      T  #dwPTR1;
      L  #dwOff;
      L  #dwPTR2;
      +D;
      T  #dwPTR2;

	L 1; 						//Verbindung 10 PCU-NR eintragen
    	T  DBB[#dwPTR1];
	T  DBB[#dwPTR2];
      L  #dwOff;
      L  #dwPTR1;
      +D;
      T  #dwPTR1;
      L  #dwOff;
      L  #dwPTR2;
      +D;
      T  #dwPTR2;

	L 2; 						//Verbindung 11 PCU-NR eintragen
    	T  DBB[#dwPTR1];
	T  DBB[#dwPTR2];
      L  #dwOff;
      L  #dwPTR1;
      +D;
      T  #dwPTR1;
      L  #dwOff;
      L  #dwPTR2;
      +D;
      T  #dwPTR2;

	L 3; 						//Verbindung 12 PCU-NR eintragen
    	T  DBB[#dwPTR1];
	T  DBB[#dwPTR2];
      L  #dwOff;
      L  #dwPTR1;
      +D;
      T  #dwPTR1;
      L  #dwOff;
      L  #dwPTR2;
      +D;
      T  #dwPTR2;

	L 4; 						//Verbindung 13 PCU-NR eintragen
    	T  DBB[#dwPTR1];
	T  DBB[#dwPTR2];
      L  #dwOff;
      L  #dwPTR1;
      +D;
      T  #dwPTR1;
      L  #dwOff;
      L  #dwPTR2;
      +D;
      T  #dwPTR2;

	L 5; 						//Verbindung 14 PCU-NR eintragen
    	T  DBB[#dwPTR1];
	T  DBB[#dwPTR2];
      L  #dwOff;
      L  #dwPTR1;
      +D;
      T  #dwPTR1;
      L  #dwOff;
      L  #dwPTR2;
      +D;
      T  #dwPTR2;

	L 6; 						//Verbindung 15 PCU-NR eintragen
    	T  DBB[#dwPTR1];
	T  DBB[#dwPTR2];
      L  #dwOff;
      L  #dwPTR1;
      +D;
      T  #dwPTR1;
      L  #dwOff;
      L  #dwPTR2;
      +D;
      T  #dwPTR2;
	spa Lo20;

AS12:	L 6; 							//Verbindung 1 PCU-NR eintragen
    	T  DBB[#dwPTR1];
	T  DBB[#dwPTR2];
      L  #dwOff;
      L  #dwPTR1;
      +D;
      T  #dwPTR1;
      L  #dwOff;
      L  #dwPTR2;
      +D;
      T  #dwPTR2;

	L 7; 							//Verbindung 2 PCU-NR eintragen
    	T  DBB[#dwPTR1];
	T  DBB[#dwPTR2];
      L  #dwOff;
      L  #dwPTR1;
      +D;
      T  #dwPTR1;
      L  #dwOff;
      L  #dwPTR2;
      +D;
      T  #dwPTR2;

	L 8; 							//Verbindung 3 PCU-NR eintragen
    	T  DBB[#dwPTR1];
	T  DBB[#dwPTR2];
      L  #dwOff;
      L  #dwPTR1;
      +D;
      T  #dwPTR1;
      L  #dwOff;
      L  #dwPTR2;
      +D;
      T  #dwPTR2;

	L 9; 							//Verbindung 4 PCU-NR eintragen
    	T  DBB[#dwPTR1];
	T  DBB[#dwPTR2];
      L  #dwOff;
      L  #dwPTR1;
      +D;
      T  #dwPTR1;
      L  #dwOff;
      L  #dwPTR2;
      +D;
      T  #dwPTR2;

	L 10; 							//Verbindung 5 PCU-NR eintragen
    	T  DBB[#dwPTR1];
	T  DBB[#dwPTR2];
      L  #dwOff;
      L  #dwPTR1;
      +D;
      T  #dwPTR1;
      L  #dwOff;
      L  #dwPTR2;
      +D;
      T  #dwPTR2;


	L 11; 							//Verbindung 6 PCU-NR eintragen
    	T  DBB[#dwPTR1];
	T  DBB[#dwPTR2];
      L  #dwOff;
      L  #dwPTR1;
      +D;
      T  #dwPTR1;
      L  #dwOff;
      L  #dwPTR2;
      +D;
      T  #dwPTR2;

	L 16; 							//Verbindung 7 PCU-NR eintragen
    	T  DBB[#dwPTR1];
	T  DBB[#dwPTR2];
      L  #dwOff;
      L  #dwPTR1;
      +D;
      T  #dwPTR1;
      L  #dwOff;
      L  #dwPTR2;
      +D;
      T  #dwPTR2;

	L 13; 							//Verbindung 8  PCU-NR eintragen
    	T  DBB[#dwPTR1];
	T  DBB[#dwPTR2];
      L  #dwOff;
      L  #dwPTR1;
      +D;
      T  #dwPTR1;
      L  #dwOff;
      L  #dwPTR2;
      +D;
      T  #dwPTR2;

	L 14; 						//Verbindung 9 PCU-NR eintragen
    	T  DBB[#dwPTR1];
	T  DBB[#dwPTR2];
      L  #dwOff;
      L  #dwPTR1;
      +D;
      T  #dwPTR1;
      L  #dwOff;
      L  #dwPTR2;
      +D;
      T  #dwPTR2;

	L 15; 						//Verbindung 10 PCU-NR eintragen
    	T  DBB[#dwPTR1];
	T  DBB[#dwPTR2];
      L  #dwOff;
      L  #dwPTR1;
      +D;
      T  #dwPTR1;
      L  #dwOff;
      L  #dwPTR2;
      +D;
      T  #dwPTR2;

	L 1; 						//Verbindung 11 PCU-NR eintragen
    	T  DBB[#dwPTR1];
	T  DBB[#dwPTR2];
      L  #dwOff;
      L  #dwPTR1;
      +D;
      T  #dwPTR1;
      L  #dwOff;
      L  #dwPTR2;
      +D;
      T  #dwPTR2;

	L 2; 						//Verbindung 12 PCU-NR eintragen
    	T  DBB[#dwPTR1];
	T  DBB[#dwPTR2];
      L  #dwOff;
      L  #dwPTR1;
      +D;
      T  #dwPTR1;
      L  #dwOff;
      L  #dwPTR2;
      +D;
      T  #dwPTR2;

	L 3; 						//Verbindung 13 PCU-NR eintragen
    	T  DBB[#dwPTR1];
	T  DBB[#dwPTR2];
      L  #dwOff;
      L  #dwPTR1;
      +D;
      T  #dwPTR1;
      L  #dwOff;
      L  #dwPTR2;
      +D;
      T  #dwPTR2;

	L 4; 						//Verbindung 14 PCU-NR eintragen
    	T  DBB[#dwPTR1];
	T  DBB[#dwPTR2];
      L  #dwOff;
      L  #dwPTR1;
      +D;
      T  #dwPTR1;
      L  #dwOff;
      L  #dwPTR2;
      +D;
      T  #dwPTR2;

	L 5; 						//Verbindung 15 PCU-NR eintragen
    	T  DBB[#dwPTR1];
	T  DBB[#dwPTR2];
      L  #dwOff;
      L  #dwPTR1;
      +D;
      T  #dwPTR1;
      L  #dwOff;
      L  #dwPTR2;
      +D;
      T  #dwPTR2;
	spa Lo20;

AS13:	L 5; 							//Verbindung 1 PCU-NR eintragen
    	T  DBB[#dwPTR1];
	T  DBB[#dwPTR2];
      L  #dwOff;
      L  #dwPTR1;
      +D;
      T  #dwPTR1;
      L  #dwOff;
      L  #dwPTR2;
      +D;
      T  #dwPTR2;

	L 6; 							//Verbindung 2 PCU-NR eintragen
    	T  DBB[#dwPTR1];
	T  DBB[#dwPTR2];
      L  #dwOff;
      L  #dwPTR1;
      +D;
      T  #dwPTR1;
      L  #dwOff;
      L  #dwPTR2;
      +D;
      T  #dwPTR2;

	L 7; 							//Verbindung 3 PCU-NR eintragen
    	T  DBB[#dwPTR1];
	T  DBB[#dwPTR2];
      L  #dwOff;
      L  #dwPTR1;
      +D;
      T  #dwPTR1;
      L  #dwOff;
      L  #dwPTR2;
      +D;
      T  #dwPTR2;

	L 8; 							//Verbindung 4 PCU-NR eintragen
    	T  DBB[#dwPTR1];
	T  DBB[#dwPTR2];
      L  #dwOff;
      L  #dwPTR1;
      +D;
      T  #dwPTR1;
      L  #dwOff;
      L  #dwPTR2;
      +D;
      T  #dwPTR2;

	L 9; 							//Verbindung 5 PCU-NR eintragen
    	T  DBB[#dwPTR1];
	T  DBB[#dwPTR2];
      L  #dwOff;
      L  #dwPTR1;
      +D;
      T  #dwPTR1;
      L  #dwOff;
      L  #dwPTR2;
      +D;
      T  #dwPTR2;


	L 10; 							//Verbindung 6 PCU-NR eintragen
    	T  DBB[#dwPTR1];
	T  DBB[#dwPTR2];
      L  #dwOff;
      L  #dwPTR1;
      +D;
      T  #dwPTR1;
      L  #dwOff;
      L  #dwPTR2;
      +D;
      T  #dwPTR2;

	L 11; 							//Verbindung 7 PCU-NR eintragen
    	T  DBB[#dwPTR1];
	T  DBB[#dwPTR2];
      L  #dwOff;
      L  #dwPTR1;
      +D;
      T  #dwPTR1;
      L  #dwOff;
      L  #dwPTR2;
      +D;
      T  #dwPTR2;

	L 12; 							//Verbindung 8  PCU-NR eintragen
    	T  DBB[#dwPTR1];
	T  DBB[#dwPTR2];
      L  #dwOff;
      L  #dwPTR1;
      +D;
      T  #dwPTR1;
      L  #dwOff;
      L  #dwPTR2;
      +D;
      T  #dwPTR2;

	L 16; 						//Verbindung 9 PCU-NR eintragen
    	T  DBB[#dwPTR1];
	T  DBB[#dwPTR2];
      L  #dwOff;
      L  #dwPTR1;
      +D;
      T  #dwPTR1;
      L  #dwOff;
      L  #dwPTR2;
      +D;
      T  #dwPTR2;

	L 14; 						//Verbindung 10 PCU-NR eintragen
    	T  DBB[#dwPTR1];
	T  DBB[#dwPTR2];
      L  #dwOff;
      L  #dwPTR1;
      +D;
      T  #dwPTR1;
      L  #dwOff;
      L  #dwPTR2;
      +D;
      T  #dwPTR2;

	L 15; 						//Verbindung 11 PCU-NR eintragen
    	T  DBB[#dwPTR1];
	T  DBB[#dwPTR2];
      L  #dwOff;
      L  #dwPTR1;
      +D;
      T  #dwPTR1;
      L  #dwOff;
      L  #dwPTR2;
      +D;
      T  #dwPTR2;

	L 1; 						//Verbindung 12 PCU-NR eintragen
    	T  DBB[#dwPTR1];
	T  DBB[#dwPTR2];
      L  #dwOff;
      L  #dwPTR1;
      +D;
      T  #dwPTR1;
      L  #dwOff;
      L  #dwPTR2;
      +D;
      T  #dwPTR2;

	L 2; 						//Verbindung 13 PCU-NR eintragen
    	T  DBB[#dwPTR1];
	T  DBB[#dwPTR2];
      L  #dwOff;
      L  #dwPTR1;
      +D;
      T  #dwPTR1;
      L  #dwOff;
      L  #dwPTR2;
      +D;
      T  #dwPTR2;

	L 3; 						//Verbindung 14 PCU-NR eintragen
    	T  DBB[#dwPTR1];
	T  DBB[#dwPTR2];
      L  #dwOff;
      L  #dwPTR1;
      +D;
      T  #dwPTR1;
      L  #dwOff;
      L  #dwPTR2;
      +D;
      T  #dwPTR2;

	L 4; 						//Verbindung 15 PCU-NR eintragen
    	T  DBB[#dwPTR1];
	T  DBB[#dwPTR2];
      L  #dwOff;
      L  #dwPTR1;
      +D;
      T  #dwPTR1;
      L  #dwOff;
      L  #dwPTR2;
      +D;
      T  #dwPTR2;
	spa Lo20;

AS14:	L 4; 							//Verbindung 1 PCU-NR eintragen
    	T  DBB[#dwPTR1];
	T  DBB[#dwPTR2];
      L  #dwOff;
      L  #dwPTR1;
      +D;
      T  #dwPTR1;
      L  #dwOff;
      L  #dwPTR2;
      +D;
      T  #dwPTR2;

	L 5; 							//Verbindung 2 PCU-NR eintragen
    	T  DBB[#dwPTR1];
	T  DBB[#dwPTR2];
      L  #dwOff;
      L  #dwPTR1;
      +D;
      T  #dwPTR1;
      L  #dwOff;
      L  #dwPTR2;
      +D;
      T  #dwPTR2;

	L 6; 							//Verbindung 3 PCU-NR eintragen
    	T  DBB[#dwPTR1];
	T  DBB[#dwPTR2];
      L  #dwOff;
      L  #dwPTR1;
      +D;
      T  #dwPTR1;
      L  #dwOff;
      L  #dwPTR2;
      +D;
      T  #dwPTR2;

	L 7; 							//Verbindung 4 PCU-NR eintragen
    	T  DBB[#dwPTR1];
	T  DBB[#dwPTR2];
      L  #dwOff;
      L  #dwPTR1;
      +D;
      T  #dwPTR1;
      L  #dwOff;
      L  #dwPTR2;
      +D;
      T  #dwPTR2;

	L 8; 							//Verbindung 5 PCU-NR eintragen
    	T  DBB[#dwPTR1];
	T  DBB[#dwPTR2];
      L  #dwOff;
      L  #dwPTR1;
      +D;
      T  #dwPTR1;
      L  #dwOff;
      L  #dwPTR2;
      +D;
      T  #dwPTR2;


	L 9; 							//Verbindung 6 PCU-NR eintragen
    	T  DBB[#dwPTR1];
	T  DBB[#dwPTR2];
      L  #dwOff;
      L  #dwPTR1;
      +D;
      T  #dwPTR1;
      L  #dwOff;
      L  #dwPTR2;
      +D;
      T  #dwPTR2;

	L 10; 							//Verbindung 7 PCU-NR eintragen
    	T  DBB[#dwPTR1];
	T  DBB[#dwPTR2];
      L  #dwOff;
      L  #dwPTR1;
      +D;
      T  #dwPTR1;
      L  #dwOff;
      L  #dwPTR2;
      +D;
      T  #dwPTR2;

	L 11; 							//Verbindung 8  PCU-NR eintragen
    	T  DBB[#dwPTR1];
	T  DBB[#dwPTR2];
      L  #dwOff;
      L  #dwPTR1;
      +D;
      T  #dwPTR1;
      L  #dwOff;
      L  #dwPTR2;
      +D;
      T  #dwPTR2;

	L 12; 						//Verbindung 9 PCU-NR eintragen
    	T  DBB[#dwPTR1];
	T  DBB[#dwPTR2];
      L  #dwOff;
      L  #dwPTR1;
      +D;
      T  #dwPTR1;
      L  #dwOff;
      L  #dwPTR2;
      +D;
      T  #dwPTR2;

	L 13; 						//Verbindung 10 PCU-NR eintragen
    	T  DBB[#dwPTR1];
	T  DBB[#dwPTR2];
      L  #dwOff;
      L  #dwPTR1;
      +D;
      T  #dwPTR1;
      L  #dwOff;
      L  #dwPTR2;
      +D;
      T  #dwPTR2;

	L 16; 						//Verbindung 11 PCU-NR eintragen
    	T  DBB[#dwPTR1];
	T  DBB[#dwPTR2];
      L  #dwOff;
      L  #dwPTR1;
      +D;
      T  #dwPTR1;
      L  #dwOff;
      L  #dwPTR2;
      +D;
      T  #dwPTR2;

	L 15; 						//Verbindung 12 PCU-NR eintragen
    	T  DBB[#dwPTR1];
	T  DBB[#dwPTR2];
      L  #dwOff;
      L  #dwPTR1;
      +D;
      T  #dwPTR1;
      L  #dwOff;
      L  #dwPTR2;
      +D;
      T  #dwPTR2;

	L 1; 						//Verbindung 13 PCU-NR eintragen
    	T  DBB[#dwPTR1];
	T  DBB[#dwPTR2];
      L  #dwOff;
      L  #dwPTR1;
      +D;
      T  #dwPTR1;
      L  #dwOff;
      L  #dwPTR2;
      +D;
      T  #dwPTR2;

	L 2; 						//Verbindung 14 PCU-NR eintragen
    	T  DBB[#dwPTR1];
	T  DBB[#dwPTR2];
      L  #dwOff;
      L  #dwPTR1;
      +D;
      T  #dwPTR1;
      L  #dwOff;
      L  #dwPTR2;
      +D;
      T  #dwPTR2;

	L 3; 						//Verbindung 15 PCU-NR eintragen
    	T  DBB[#dwPTR1];
	T  DBB[#dwPTR2];
      L  #dwOff;
      L  #dwPTR1;
      +D;
      T  #dwPTR1;
      L  #dwOff;
      L  #dwPTR2;
      +D;
      T  #dwPTR2;
	spa Lo20;

AS15:	L 3; 							//Verbindung 1 PCU-NR eintragen
    	T  DBB[#dwPTR1];
	T  DBB[#dwPTR2];
      L  #dwOff;
      L  #dwPTR1;
      +D;
      T  #dwPTR1;
      L  #dwOff;
      L  #dwPTR2;
      +D;
      T  #dwPTR2;

	L 4; 							//Verbindung 2 PCU-NR eintragen
    	T  DBB[#dwPTR1];
	T  DBB[#dwPTR2];
      L  #dwOff;
      L  #dwPTR1;
      +D;
      T  #dwPTR1;
      L  #dwOff;
      L  #dwPTR2;
      +D;
      T  #dwPTR2;

	L 5; 							//Verbindung 3 PCU-NR eintragen
    	T  DBB[#dwPTR1];
	T  DBB[#dwPTR2];
      L  #dwOff;
      L  #dwPTR1;
      +D;
      T  #dwPTR1;
      L  #dwOff;
      L  #dwPTR2;
      +D;
      T  #dwPTR2;

	L 6; 							//Verbindung 4 PCU-NR eintragen
    	T  DBB[#dwPTR1];
	T  DBB[#dwPTR2];
      L  #dwOff;
      L  #dwPTR1;
      +D;
      T  #dwPTR1;
      L  #dwOff;
      L  #dwPTR2;
      +D;
      T  #dwPTR2;

	L 7; 							//Verbindung 5 PCU-NR eintragen
    	T  DBB[#dwPTR1];
	T  DBB[#dwPTR2];
      L  #dwOff;
      L  #dwPTR1;
      +D;
      T  #dwPTR1;
      L  #dwOff;
      L  #dwPTR2;
      +D;
      T  #dwPTR2;


	L 8; 							//Verbindung 6 PCU-NR eintragen
    	T  DBB[#dwPTR1];
	T  DBB[#dwPTR2];
      L  #dwOff;
      L  #dwPTR1;
      +D;
      T  #dwPTR1;
      L  #dwOff;
      L  #dwPTR2;
      +D;
      T  #dwPTR2;

	L 9; 							//Verbindung 7 PCU-NR eintragen
    	T  DBB[#dwPTR1];
	T  DBB[#dwPTR2];
      L  #dwOff;
      L  #dwPTR1;
      +D;
      T  #dwPTR1;
      L  #dwOff;
      L  #dwPTR2;
      +D;
      T  #dwPTR2;

	L 10; 							//Verbindung 8  PCU-NR eintragen
    	T  DBB[#dwPTR1];
	T  DBB[#dwPTR2];
      L  #dwOff;
      L  #dwPTR1;
      +D;
      T  #dwPTR1;
      L  #dwOff;
      L  #dwPTR2;
      +D;
      T  #dwPTR2;

	L 11; 						//Verbindung 9 PCU-NR eintragen
    	T  DBB[#dwPTR1];
	T  DBB[#dwPTR2];
      L  #dwOff;
      L  #dwPTR1;
      +D;
      T  #dwPTR1;
      L  #dwOff;
      L  #dwPTR2;
      +D;
      T  #dwPTR2;

	L 12; 						//Verbindung 10 PCU-NR eintragen
    	T  DBB[#dwPTR1];
	T  DBB[#dwPTR2];
      L  #dwOff;
      L  #dwPTR1;
      +D;
      T  #dwPTR1;
      L  #dwOff;
      L  #dwPTR2;
      +D;
      T  #dwPTR2;

	L 13; 						//Verbindung 11 PCU-NR eintragen
    	T  DBB[#dwPTR1];
	T  DBB[#dwPTR2];
      L  #dwOff;
      L  #dwPTR1;
      +D;
      T  #dwPTR1;
      L  #dwOff;
      L  #dwPTR2;
      +D;
      T  #dwPTR2;

	L 14; 						//Verbindung 12 PCU-NR eintragen
    	T  DBB[#dwPTR1];
	T  DBB[#dwPTR2];
      L  #dwOff;
      L  #dwPTR1;
      +D;
      T  #dwPTR1;
      L  #dwOff;
      L  #dwPTR2;
      +D;
      T  #dwPTR2;

	L 16; 						//Verbindung 13 PCU-NR eintragen
    	T  DBB[#dwPTR1];
	T  DBB[#dwPTR2];
      L  #dwOff;
      L  #dwPTR1;
      +D;
      T  #dwPTR1;
      L  #dwOff;
      L  #dwPTR2;
      +D;
      T  #dwPTR2;

	L 1; 						//Verbindung 14 PCU-NR eintragen
    	T  DBB[#dwPTR1];
	T  DBB[#dwPTR2];
      L  #dwOff;
      L  #dwPTR1;
      +D;
      T  #dwPTR1;
      L  #dwOff;
      L  #dwPTR2;
      +D;
      T  #dwPTR2;

	L 2; 						//Verbindung 15 PCU-NR eintragen
    	T  DBB[#dwPTR1];
	T  DBB[#dwPTR2];
      L  #dwOff;
      L  #dwPTR1;
      +D;
      T  #dwPTR1;
      L  #dwOff;
      L  #dwPTR2;
      +D;
      T  #dwPTR2;
	spa Lo20;

AS16:	L 9; 							//Verbindung 1 PCU-NR eintragen
    	T  DBB[#dwPTR1];
	T  DBB[#dwPTR2];
      L  #dwOff;
      L  #dwPTR1;
      +D;
      T  #dwPTR1;
      L  #dwOff;
      L  #dwPTR2;
      +D;
      T  #dwPTR2;

	L 2; 							//Verbindung 2 PCU-NR eintragen
    	T  DBB[#dwPTR1];
	T  DBB[#dwPTR2];
      L  #dwOff;
      L  #dwPTR1;
      +D;
      T  #dwPTR1;
      L  #dwOff;
      L  #dwPTR2;
      +D;
      T  #dwPTR2;

	L 10; 							//Verbindung 3 PCU-NR eintragen
    	T  DBB[#dwPTR1];
	T  DBB[#dwPTR2];
      L  #dwOff;
      L  #dwPTR1;
      +D;
      T  #dwPTR1;
      L  #dwOff;
      L  #dwPTR2;
      +D;
      T  #dwPTR2;

	L 3; 							//Verbindung 4 PCU-NR eintragen
    	T  DBB[#dwPTR1];
	T  DBB[#dwPTR2];
      L  #dwOff;
      L  #dwPTR1;
      +D;
      T  #dwPTR1;
      L  #dwOff;
      L  #dwPTR2;
      +D;
      T  #dwPTR2;

	L 11; 							//Verbindung 5 PCU-NR eintragen
    	T  DBB[#dwPTR1];
	T  DBB[#dwPTR2];
      L  #dwOff;
      L  #dwPTR1;
      +D;
      T  #dwPTR1;
      L  #dwOff;
      L  #dwPTR2;
      +D;
      T  #dwPTR2;


	L 4; 							//Verbindung 6 PCU-NR eintragen
    	T  DBB[#dwPTR1];
	T  DBB[#dwPTR2];
      L  #dwOff;
      L  #dwPTR1;
      +D;
      T  #dwPTR1;
      L  #dwOff;
      L  #dwPTR2;
      +D;
      T  #dwPTR2;

	L 12; 							//Verbindung 7 PCU-NR eintragen
    	T  DBB[#dwPTR1];
	T  DBB[#dwPTR2];
      L  #dwOff;
      L  #dwPTR1;
      +D;
      T  #dwPTR1;
      L  #dwOff;
      L  #dwPTR2;
      +D;
      T  #dwPTR2;

	L 5; 							//Verbindung 8  PCU-NR eintragen
    	T  DBB[#dwPTR1];
	T  DBB[#dwPTR2];
      L  #dwOff;
      L  #dwPTR1;
      +D;
      T  #dwPTR1;
      L  #dwOff;
      L  #dwPTR2;
      +D;
      T  #dwPTR2;

	L 13; 						//Verbindung 9 PCU-NR eintragen
    	T  DBB[#dwPTR1];
	T  DBB[#dwPTR2];
      L  #dwOff;
      L  #dwPTR1;
      +D;
      T  #dwPTR1;
      L  #dwOff;
      L  #dwPTR2;
      +D;
      T  #dwPTR2;

	L 6; 						//Verbindung 10 PCU-NR eintragen
    	T  DBB[#dwPTR1];
	T  DBB[#dwPTR2];
      L  #dwOff;
      L  #dwPTR1;
      +D;
      T  #dwPTR1;
      L  #dwOff;
      L  #dwPTR2;
      +D;
      T  #dwPTR2;

	L 14; 						//Verbindung 11 PCU-NR eintragen
    	T  DBB[#dwPTR1];
	T  DBB[#dwPTR2];
      L  #dwOff;
      L  #dwPTR1;
      +D;
      T  #dwPTR1;
      L  #dwOff;
      L  #dwPTR2;
      +D;
      T  #dwPTR2;

	L 7; 						//Verbindung 12 PCU-NR eintragen
    	T  DBB[#dwPTR1];
	T  DBB[#dwPTR2];
      L  #dwOff;
      L  #dwPTR1;
      +D;
      T  #dwPTR1;
      L  #dwOff;
      L  #dwPTR2;
      +D;
      T  #dwPTR2;

	L 15; 						//Verbindung 13 PCU-NR eintragen
    	T  DBB[#dwPTR1];
	T  DBB[#dwPTR2];
      L  #dwOff;
      L  #dwPTR1;
      +D;
      T  #dwPTR1;
      L  #dwOff;
      L  #dwPTR2;
      +D;
      T  #dwPTR2;

	L 8; 						//Verbindung 14 PCU-NR eintragen
    	T  DBB[#dwPTR1];
	T  DBB[#dwPTR2];
      L  #dwOff;
      L  #dwPTR1;
      +D;
      T  #dwPTR1;
      L  #dwOff;
      L  #dwPTR2;
      +D;
      T  #dwPTR2;

	L 1; 						//Verbindung 15 PCU-NR eintragen
    	T  DBB[#dwPTR1];
	T  DBB[#dwPTR2];
      L  #dwOff;
      L  #dwPTR1;
      +D;
      T  #dwPTR1;
      L  #dwOff;
      L  #dwPTR2;
      +D;
      T  #dwPTR2;
	spa Lo20;



//Schleife um alle Verbindungen zu Bearbeiten
Lo20: L "XC_VERB_SR".iAct;
Lo22:	T  #iAct;

	L  "XC_VERB_SR".iLen;		//Anzahl
      T #iLoop;

      L   #iAct;
	+  -1;
	L   "XC_VERB_SR".iLen;
      *I;
	L   "XC_VERB_SR".iOffset;
	+I;
	SLD 3;
	T #dwPTR1;		//Bereichszeiger

	LAR1 p#20.0;       //Pionter auf uVERB in den lokalen Daten
	auf  "XC_VERB_SR";

//Schleife um Daten in lokale Variable Byteweise umzuladen
	L  "XC_VERB_SR".iLen;		//Anzahl der Bytes
Lo21: T #iLoop;

      L DBB[#dwPTR1];		//Wert aus DB holen
	T LB [AR1,p#0.0];		//Wert in uVERB eintragen

	+AR1 p#1.0;			//AR1 um 1Bytes erhoehen
	l  #dwPTR1;			//Zeiger fuer DB-Datenwort erhoehen
	L 8;
	+D;
	T #dwPTR1;
	L   #iLoop;			//Schleifenzaehler erniedrigen und zum Anfang
	LOOP Lo21;

//Werte eintragen	dh. Verbindung 15 ... 1

	L 986;					//Sendepuffer DB
      T  uVerb.iSendDB;
	L 987;					//Empfangspuffer DB
      T  uVerb.iRecvDB;
	L 240;					//Laenge der Puffer
      T  uVerb.iLEN;

	L   #iAct;
	+  -1;
	L 240;
	*I;
	T  uVerb.iSendDW;			//Sendepuffer Anfang
	T  uVerb.iRecvDW;			//Empfangspuffer Anfang

	on m 0.0;
	o m 0.0;
	S  uVerb.boS7;					//Kennungen Koppelpartner = S7 setzen
	S  uVerb.boAS7;
	S  uVerb.boRS7;
	S  uVerb.boAAktiv;

	R  uVerb.boS5;					//Kennungen Koppelpartner = S5 Ruecksetzen
	R  uVerb.boAS5;
	R  uVerb.boRS5;
	R  uVerb.boRAktiv;

	l  w#16#3e80;
	T  uVerb.wLADDR;				//Adresse der Hardware
	T  uVerb.wALADDR;			//Adresse der Hardware
	T  uVerb.wRLADDR;			//Adresse der Hardware


	L 0;
	T  uVerb.bRPCU;				//PCU-Nummer

	L   #iAct;
      + -1;
	L 2;
	*I;
	L   "XC_VERB_SR".bOffID;
      +I;
	T  uVerb.iID;				//Hardware ID-Nummer
	T  uVerb.iAID;				//Hardware ID-Nummer
	T  uVerb.iRID;				//Hardware ID-Nummer

      L   #iAct;
	+  -1;
	L   "XC_VERB_SR".iLen;
      *I;
	L   "XC_VERB_SR".iOffset;
	+I;
	SLD 3;
	T #dwPTR1;		//Bereichszeiger

	LAR1 p#20.0;       //Pionter auf uVERB in den lokalen Daten
	auf  "XC_VERB_SR";

//Schleife um Daten zurueck zuladen
	L  "XC_VERB_SR".iLen;		//Anzahl Bytes
Lo23: T #iLoop;

	L LB [AR1,p#0.0];		//Wert in uVERB eintragen
      T DBB[#dwPTR1];		//Wert aus DB holen

	+AR1 p#1.0;			//AR1 um 1Bytes erhoehen
	l  #dwPTR1;			//Zeiger fuer DB-Datenwort erhoehen
	L 8;
	+D;
	T #dwPTR1;
	L   #iLoop;			//Schleifenzaehler erniedrigen und zum Anfang
	LOOP Lo23;

	L  #iAct;
	LOOP Lo22;

end2: NOP 0;

NETWORK
TITLE = KOPPLUNG - Empfangen und Senden
// ===========================================================================

//**********************
//Verbindungsdaten laden
//**********************

      l iFKT;
	l 1;
	<>I;
	spb end3;

//Schleife um alle Verbindungen zu Bearbeiten
	L  "XC_VERB_SR".iAct;
	T  #iAct;

Lo32:	L  "XC_VERB_SR".iLen;		//Anzahl
      T #iLoop;

      L   #iAct;
	+  -1;
	L   "XC_VERB_SR".iLen;
      *I;
	L   "XC_VERB_SR".iOffset;
	+I;
	SLD 3;
	T #dwPTR1;		//Bereichszeiger

	LAR1 p#20.0;       //Pionter auf uVERB in den lokalen Daten
	auf  "XC_VERB_SR";

//Schleife um Daten in lokale Variable umzuladen
	L  "XC_VERB_SR".iLen;		//Anzahl der Bytes
Lo31: T #iLoop;

      L DBB[#dwPTR1];		//Wert aus DB holen
	T LB [AR1,p#0.0];		//Wert in uVERB eintragen

	+AR1 p#1.0;			//AR1 um 1Bytes erhoehen
	l  #dwPTR1;			//Zeiger fuer DB-Datenwort erhoehen
	L 8;
	+D;
	T #dwPTR1;
	L   #iLoop;			//Schleifenzaehler erniedrigen und zum Anfang
	LOOP Lo31;


//********************
//Empfang
//********************

//Pruefen ob Empfangspuffer frei ist
      U   #uVerb.boREPU;
 	spb Send;

	L	uVerb.iID;
      + 1;
	T #iID;
	L	uVerb.wLADDR;
	T #wLADDR;

	L	uVerb.iLEN;
	T #iLEN;

//Pionter fuer den Empfangspuffer zusammenstellen
//Any-Pointer:
//Byte 0	: S7-Typ 		= 16=10H
//Byte 1	: Datentyp		= 02=Byte
//Byte 2/3	: Wiederholungsfaktor
//Byte 4/5	: DB-Nummer
//Byte 6-9	: Bereichszeiger

	L uVerb.iLEN;	//Anzahl 120 DW
	T LW 12;
      L uVerb.iRecvDB;	//DB-NR
	T LW 14;
	L  uVerb.iRecvDW;
	SLD 3;
	T LD 16;		//Bereichszeiger dh. DW im DB
      L 8;
	T LB 16;		//Kennung DB

//Datenempfang in den Empfangspuffer eintragen
      call "AG_LRECV"
      (
		ID		:= #iID,
		LADDR		:= #wLADDR,
		RECV		:= #anyZIEL,
		NDR		:= #boNDR,
		ERROR		:= #boERROR,
		STATUS	:= #wSTATUS,
		LEN		:= #iLEN
      );

//Ergebnise wieder zuruecksichern
      U #boNDR;
      = uVerb.boRecvNDR;
	U #boERROR;
      = uVerb.boRecvERROR;
	L #wSTATUS;
     	T uVerb.wRecvSTATUS;
	L #iLEN;
      T uVerb.iRecvLEN;

//Pruefen ob Puffer beschrieben wurde
	UN #boNDR;
	spb Send;
	S  uVerb.boREPU;				//Kennung Empfangspuffer belegt dh. Daten entsorgen
	L  uVerb.bRecvCount;			//Empfangszaehler erhoehen
	INC 1;
	T  uVerb.bRecvCount;

//****************************
//Senden
//****************************


//Pruefen ob Sendepuffer belegt ist

Send:	L	uVerb.iID;
 	T #iID;

	L	uVerb.wLADDR;
	T #wLADDR;

	L	uVerb.iLEN;
	T #iLEN;

//Pionter fuer den Sendepuffer zusammenstellen
//Any-Pointer:
//Byte 0	: S7-Typ 		= 16=10H
//Byte 1	: Datentyp		= 02=Byte
//Byte 2/3	: Wiederholungsfaktor
//Byte 4/5	: DB-Nummer
//Byte 6-9	: Bereichszeiger

	L uVerb.iLEN;	//Anzahl 120 DW
	T LW 2;
      L uVerb.iSendDB;	//DB-NR
	T LW 4;
	L  uVerb.iSendDW;
	SLD 3;
	T LD 6;		//Bereichszeiger dh. DW im DB
      L 8;
	T LB 6;		//Kennung DB


//Daten aus dem Sendepuffer senden

	U	uVerb.boSEPU;           //Sendepuffer ist belegt dh. Senden anstossen
	=	#boSend;

	un	#boSend;
	spb	Sefe;

     call "AG_LSEND"
      (
		ACT		:= #boSend,
		ID		:= #iID,
		LADDR		:= #wLADDR,
		SEND		:= #anyQUEL,
		LEN		:= #iLEN,
		DONE		:= #boDONE,
		ERROR		:= #boERROR,
		STATUS	:= #wSTATUS
      );


//Ergebnise wieder zuruecksichern
      U #boDONE;
      = uVerb.boSendDONE;
	U #boERROR;
      = uVerb.boSendERROR;
	L #wSTATUS;
     	T uVerb.wSendSTATUS;

//Pruefen ob Puffer beschrieben wurde
Sefe:	U #boDONE;
	U #boSend;
	R  uVerb.boSEPU;				//Kennung Sendepuffer belegt dh. Daten entsorgen

//************************
//Verbindungsdaten zurueck
//************************

LA31:	L   #iAct;
	+  -1;
	L   "XC_VERB_SR".iLen;
      *I;
	L   "XC_VERB_SR".iOffset;
	+I;
	SLD 3;
	T #dwPTR1;		//Bereichszeiger

	LAR1 p#20.0;       //Pionter auf uVERB in den lokalen Daten
	auf  "XC_VERB_SR";

//Schleife um Daten zurueck zuladen
	L  "XC_VERB_SR".iLen;		//Anzahl in Bytes
Lo33: T #iLoop;

	L LB [AR1,p#0.0];		//Wert in uVERB eintragen
      T DBB[#dwPTR1];		//Wert aus DB holen

	+AR1 p#1.0;			//AR1 um 1Bytes erhoehen
	l  #dwPTR1;			//Zeiger fuer DB-Datenwort erhoehen
	L 8;
	+D;
	T #dwPTR1;
	L   #iLoop;			//Schleifenzaehler erniedrigen und zum Anfang
	LOOP Lo33;

Ne31:	L  #iAct;
       + -1;
      t  #iAct;
      l 0;
      >I;
	spb Lo32;


end3: nop 0;



NETWORK
TITLE =RECEIVE	- Empfangspuffer entsorgen
// ===========================================================================

        l iFKT;
	  l 1;
	  <>I;
	  spb end4;

//Schleife um alle Verbindungen zu Bearbeiten
 	L   "XC_VERB_SR".bRVB;
	t  #bySavVB;

	L  "XC_VERB_SR".bRVBmax;
	t #iAct;

Lo42:	nop 0;

	L  "XC_VERB_SR".iLen;		//Anzahl
      T #iLoop;

      L   "XC_VERB_SR".bRVB;
	INC 1;
	T   "XC_VERB_SR".bRVB;
	L   "XC_VERB_SR".iAct;
	<=I;
	SPB an41;
	L 1;
	T   "XC_VERB_SR".bRVB;

an41:	L	"XC_VERB_SR".bRVB;
	+  -1;
	L   "XC_VERB_SR".iLen;
      *I;
	L   "XC_VERB_SR".iOffset;
	+I;
	SLD 3;
	T #dwPTR1;		//Bereichszeiger

	LAR1 p#20.0;       //Pionter auf uVERB in den lokalen Daten
	auf  "XC_VERB_SR";

//Schleife um Daten in lokale Variable Byteweise umzuladen
	L  "XC_VERB_SR".iLen;		//Anzahl der Bytes
Lo41: T #iLoop;

      L DBB[#dwPTR1];		//Wert aus DB holen
	T LB [AR1,p#0.0];		//Wert in uVERB eintragen

	+AR1 p#1.0;			//AR1 um 1Bytes erhoehen
	l  #dwPTR1;			//Zeiger fuer DB-Datenwort erhoehen
	L 8;
	+D;
	T #dwPTR1;
	L   #iLoop;			//Schleifenzaehler erniedrigen und zum Anfang
	LOOP Lo41;

//Pruefen ob Empfangsdaten vorhanden sind
      UN   uVerb.boREPU;
      spb  Ne41;
	R    uVerb.boREPU;

      L #iAct;
	dec 1;
	t  #iAct;

	L  "XC_VERB_SR".bRVB;
	T #iret;

	CALL "FC_SR_RECV"(
               iFKT 	:=	1,
		   iVBNR	:=	#iret
				);


	L	"XC_VERB_SR".bRVB;
 	+  -1;
	L   "XC_VERB_SR".iLen;
      *I;
	L   "XC_VERB_SR".iOffset;
	+I;
	SLD 3;
	T #dwPTR1;		//Bereichszeiger

	LAR1 p#20.0;       //Pionter auf uVERB in den lokalen Daten
	auf  "XC_VERB_SR";

//Schleife um Daten zurueck zuladen
	L  "XC_VERB_SR".iLen;		//Anzahl Bytes
Lo43: T #iLoop;

	L LB [AR1,p#0.0];		//Wert in uVERB eintragen
      T DBB[#dwPTR1];		//Wert aus DB holen

	+AR1 p#1.0;			//AR1 um 1Bytes erhoehen
	l  #dwPTR1;			//Zeiger fuer DB-Datenwort erhoehen
	L 8;
	+D;
	T #dwPTR1;
	L   #iLoop;			//Schleifenzaehler erniedrigen und zum Anfang
	LOOP Lo43;

Ne41:	L  #iAct;			//Maximale Anzahl Bearbeitungen pro Zyklus abgelaufen
      l  0;
	==I;
      spb end4;
	L	"XC_VERB_SR".bRVB; //Maximal jede Verbindung einmal pruefen
	l  #bySavVB;
      <>I;
	spb Lo42;

end4: NOP 0;



NETWORK
TITLE =SEND	- Sendepuffer eintragen, Senden, Sendung ueberwachen
// ===========================================================================

        l iFKT;
	  l 1;
	  <>I;
	  spb end5;

//Schleife um alle Verbindungen zu Bearbeiten
 	L   "XC_VERB_SR".bSVB;
	t  #bySavVB;

	L  "XC_VERB_SR".bSVBmax;
	t #iAct;

Lo52:	nop 0;

	L  "XC_VERB_SR".iLen;		//Anzahl
      T #iLoop;

      L   "XC_VERB_SR".bSVB;
	INC 1;
	T   "XC_VERB_SR".bSVB;
	L   "XC_VERB_SR".iAct;
	<=I;
	SPB an51;
	L 1;
	T   "XC_VERB_SR".bSVB;

an51: L #iAct;
	dec 1;
	t  #iAct;

	L  "XC_VERB_SR".bSVB;
	T #iret;

	CALL "FC_SR_SEND"(
               iFKT 	:=	1,
		   iVBNR	:=	#iret
				);


Ne51:	L  #iAct;			//Maximale Anzahl Bearbeitungen pro Zyklus abgelaufen
      l  0;
	==I;
      spb end5;
	L	"XC_VERB_SR".bSVB; //Maximal jede Verbindung einmal pruefen
	l  #bySavVB;
      <>I;
	spb Lo52;

end5: NOP 0;


NETWORK
TITLE =TIME	- ALARM 100 ms im OB35 bearbeiten
// ===========================================================================

        l iFKT;
	  l 100;
	  <>I;
	  spb end6;
	  r #bosec;
	  r #bomin;

	  l   "XC_VERB_SR".bsec;			//100 ms Zaehler fuer Sekunde
	  inc 1;
	  t   "XC_VERB_SR".bsec;
	  l 10;
	  <>I;
	  spb  ms;
	  l 0;
	  t "XC_VERB_SR".bsec;
 	  s #bosec;

	  l "XC_VERB_SR".bmin;             //Sec - Zaehler fuer Minute
	  inc 1;
	  t   "XC_VERB_SR".bmin;
	  l 60;
	  <>I;
	  spb  ms;
	  l 0;
	  t "XC_VERB_SR".bmin;
 	  s #bomin;

ms: 	  nop 0;				//In einer Schleife alle Jobs bearbeiten
	  l 1;
	  t #iAct;

        Auf "XC_JOB_SR";

ms1:    l #iAct;
        l -1;
        +I;
        l "XC_JOB_SR".iLen ;
        *I;
	  l "XC_JOB_SR".iOffset ;
        +i;
        sld 3;
	  LAR1; 	        //Offset zum Anfang des Job-Blocks

        L  DBW[AR1,p#0.0];   //PCU = 0 dh. keine Bearbeitung
        L 0;
	  ==I;
	  spb ne60;
        o dbx[AR1,p#3.0];   //Bit 0 = Auftrag laeuft
        o dbx[AR1,p#3.2];   //Bit 2 = Verbindung fehlerhaft
	  spb er60;

  	  l dbw[AR1,p#28.0];   //Sollzeit = 0 dh. keine Bearbeitung
        l 0;
        ==I;
	  spb er60;

	  l 0;
        T  DBW[AR1,p#40.0];  //Ersatzwertzeit aus

        u  dbx[AR1,p#3.4];   //Bit 4 = 1 dh. Zeitbasis msec
	  spb ti60;
        un dbx[AR1,p#3.4];   //Bit 4 = 0 dh. Zeitbasis sec
	  un dbx[AR1,p#3.5];   //Bit 5 = 0
	  u #bosec;
        spb ti60;
        u dbx[AR1,p#3.5];   //Bit 5 = 1 dh. Zeitbasis min
	  u #bomin;
        spb ti60;
        spb er60;


ti60:   l dbw[AR1,p#30.0];   //Istzeit erhoehen   Sendezeit
        l 1;
	  +I;
        t dbw[AR1,p#30.0];   //Istzeit
	  L dbw[AR1,p#28.0];   //Sollzeit
        <I;
	  spb er60;
 	  s dbx[AR1,p#3.0];   //Bit 0 = Auftrag freigeben zum Senden

	  l 0;
        t dbw[AR1,p#30.0];   //Istzeit neu starten

er60:   nop 0;			//Ersatzwert bearbeiten
	  u  dbx[AR1,p#3.2];   //Bit 2 = 1 dh. Verbindung fehlerhaft
	  spb er61;
	  l 0;
        T  DBW[AR1,p#40.0];  //Ersatzwertzeit aus
        spb ne60;

er61:  u  dbx[AR1,p#3.4];   //Bit 4 = 1 dh. Zeitbasis msec
	  spb ti61;
        un dbx[AR1,p#3.4];   //Bit 4 = 0 dh. Zeitbasis sec
	  un dbx[AR1,p#3.5];   //Bit 5 = 0
	  u #bosec;
        spb ti61;
        u dbx[AR1,p#3.5];   //Bit 5 = 1 dh. Zeitbasis min
	  u #bomin;
        spb ti61;
        spb ne60;

ti61:   l dbw[AR1,p#38.0];   //Sollzeit = 0 dh. keine Bearbeitung
        l 0;
        ==I;
	  spb ne60;

        l dbw[AR1,p#40.0];   //Istzeit
	  L 0;
        ==I;
	  spb st61;
	  l dbw[AR1,p#40.0];   //Istzeit
	  L dbw[AR1,p#38.0];   //Sollzeit
        >I;
	  spb ne60;
st61:	  l dbw[AR1,p#40.0];   //Istzeit erhoehen Ersatzwert
        l 1;
	  +I;
        t dbw[AR1,p#40.0];   //Istzeit


ne60:   l #iAct;				//Naechsten Job anwaehlen
	  l 1;
        +i;
	  t #iAct;
	  l "XC_JOB_SR".iAct;
        <=I;
        spb ms1;

end6:   nop 0;


NETWORK
TITLE =ERSATZWERTE
// ===========================================================================
	  l iFKT;
	  l 1;
	  <>I;
	  spb end7;

 	  l "XC_VERB_SR".iPrtErsa;
        l 1;
        +I;
 	  t "XC_VERB_SR".iPrtErsa;
 	  l "XC_VERB_SR".iAct;
        <=I;
        spb la70;
        l 1;
        t "XC_VERB_SR".iPrtErsa;

la70:  l "XC_VERB_SR".iPrtErsa;
       t #iret;

	 CALL "FC_SR_ERSA"(                    //Evtl. Fehlerbits im Job setzen
               iFKT 	:=	1,
		   iVBNR	:=	#iret
				);



	 CALL "FC_SR_ERSA"(                    //Ersatzwerte umladen
               iFKT 	:=	2,
		   iVBNR	:=	#iret
				);



end7:  nop 0;

NETWORK
TITLE =KETTENSTART FUER EBENE 4 S7 - S7
// ===========================================================================

call fc 654 (			//Teilanlage starten aufgrund Tel. von S7
		iFkt	:=72		//das mit Send-DB direkt in den DB688 kommt
		);


END_FUNCTION
